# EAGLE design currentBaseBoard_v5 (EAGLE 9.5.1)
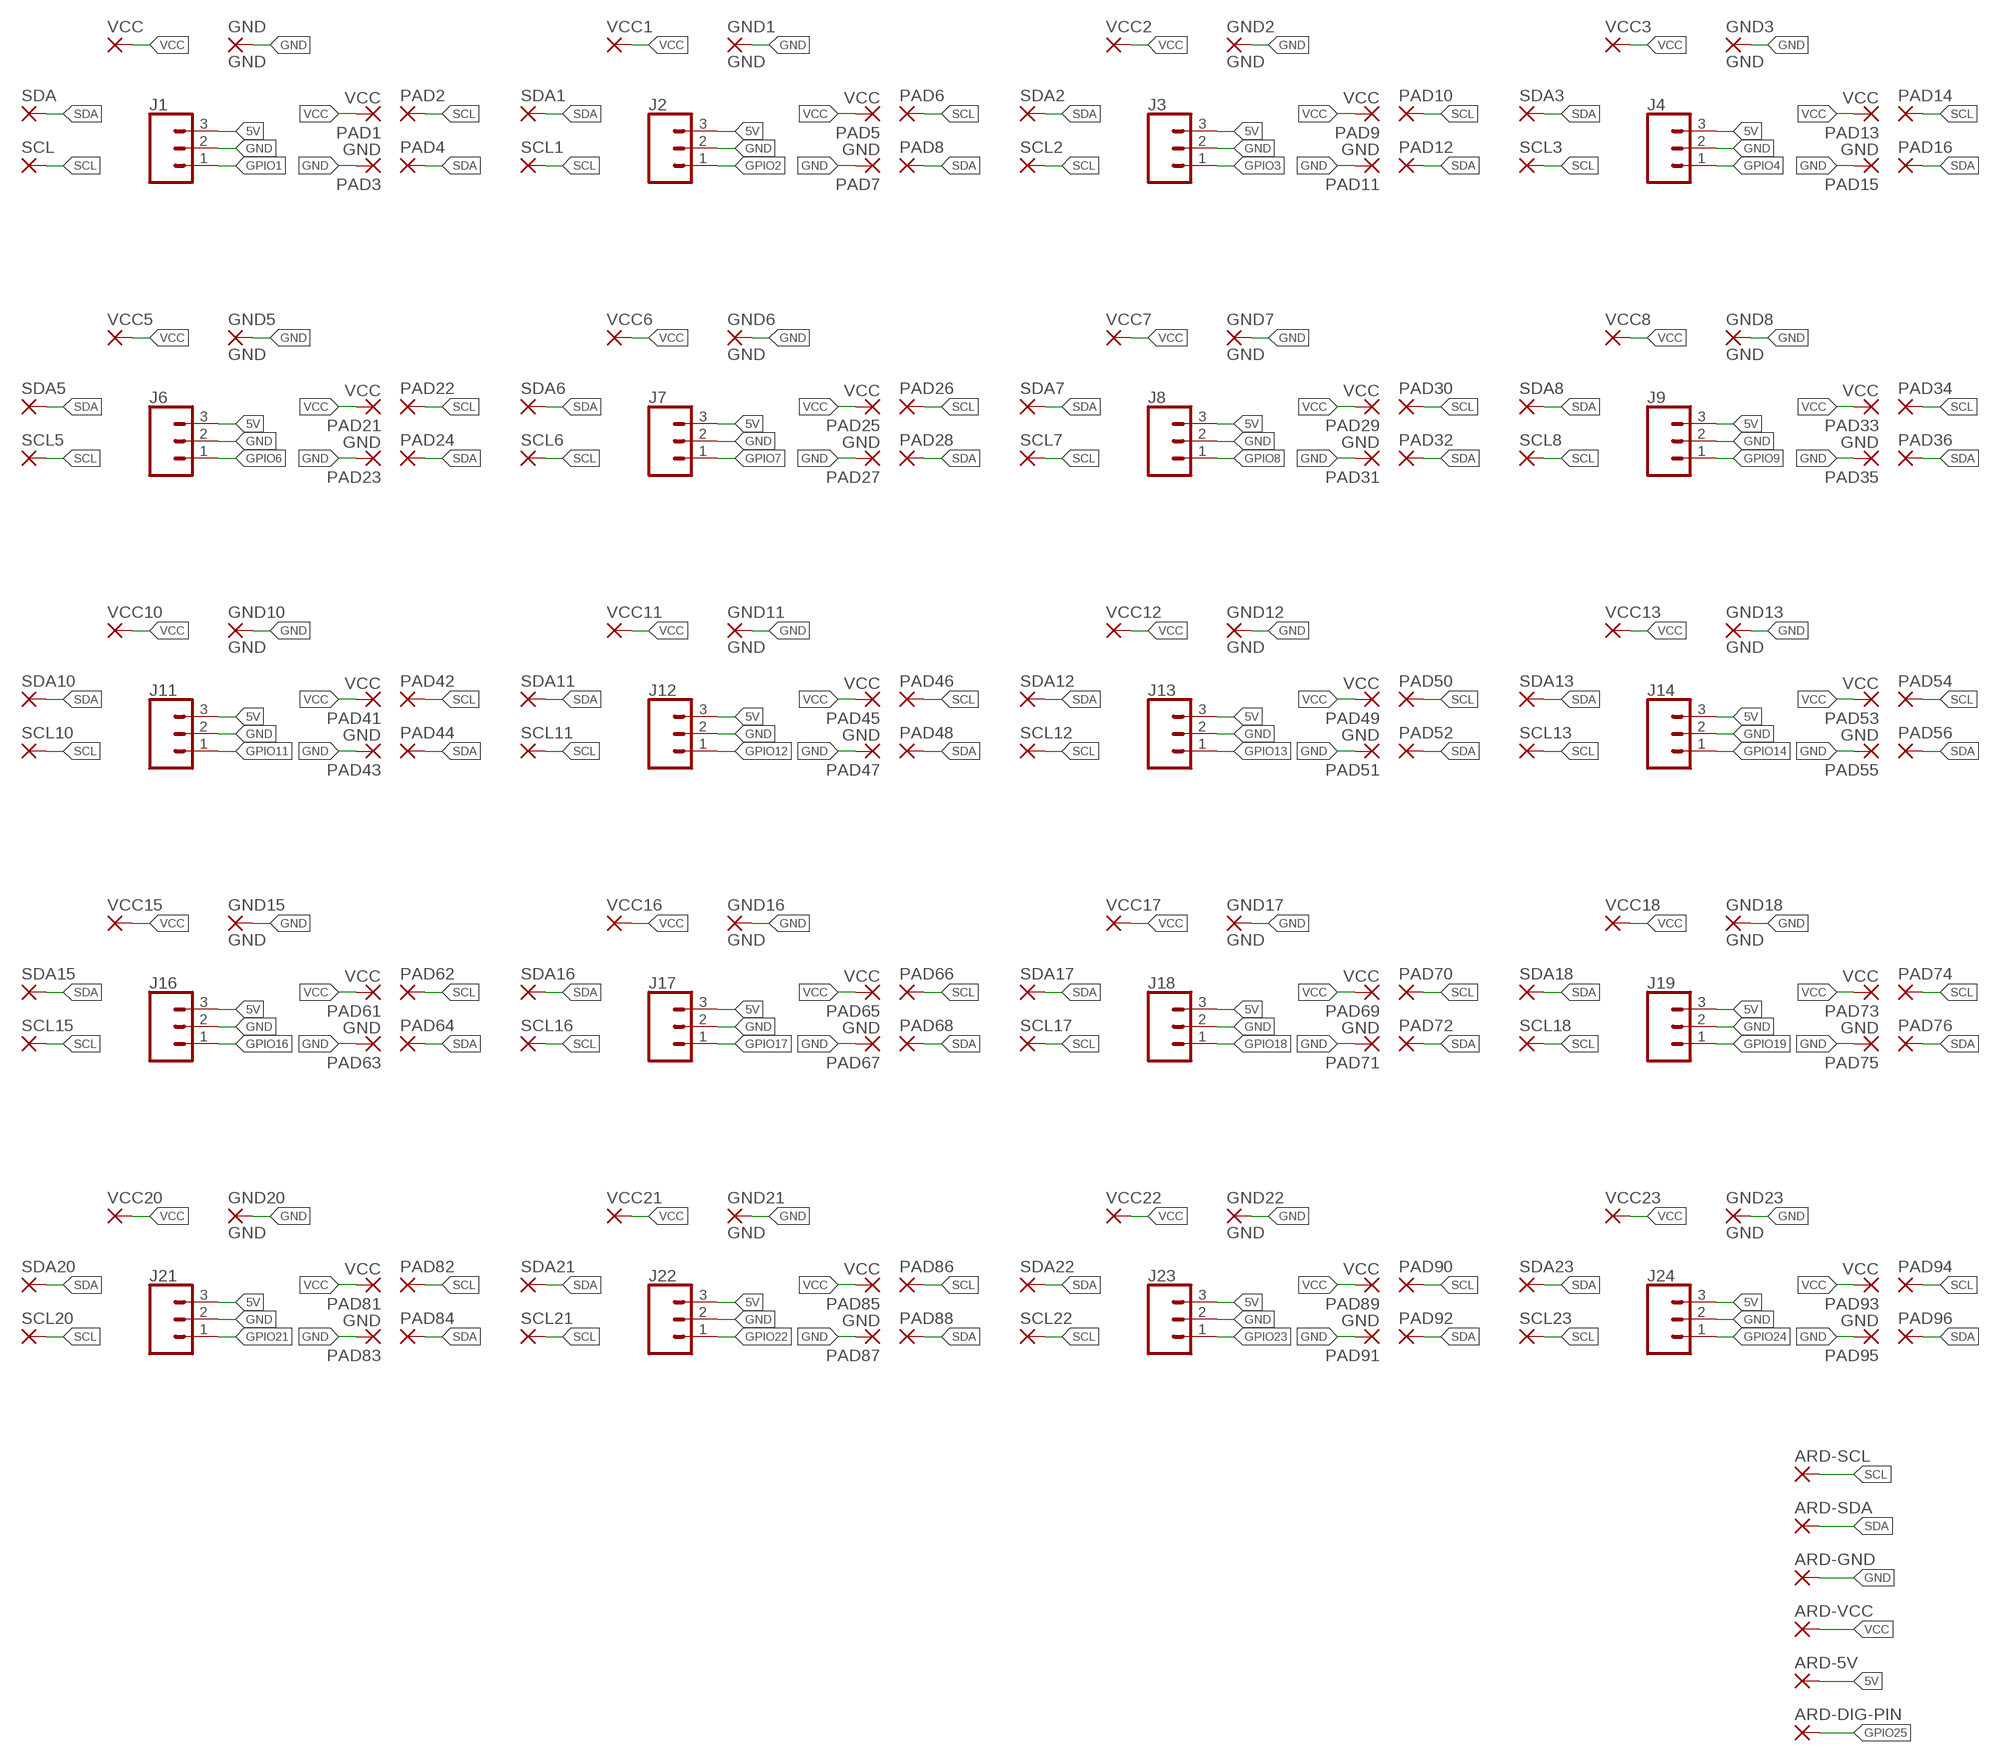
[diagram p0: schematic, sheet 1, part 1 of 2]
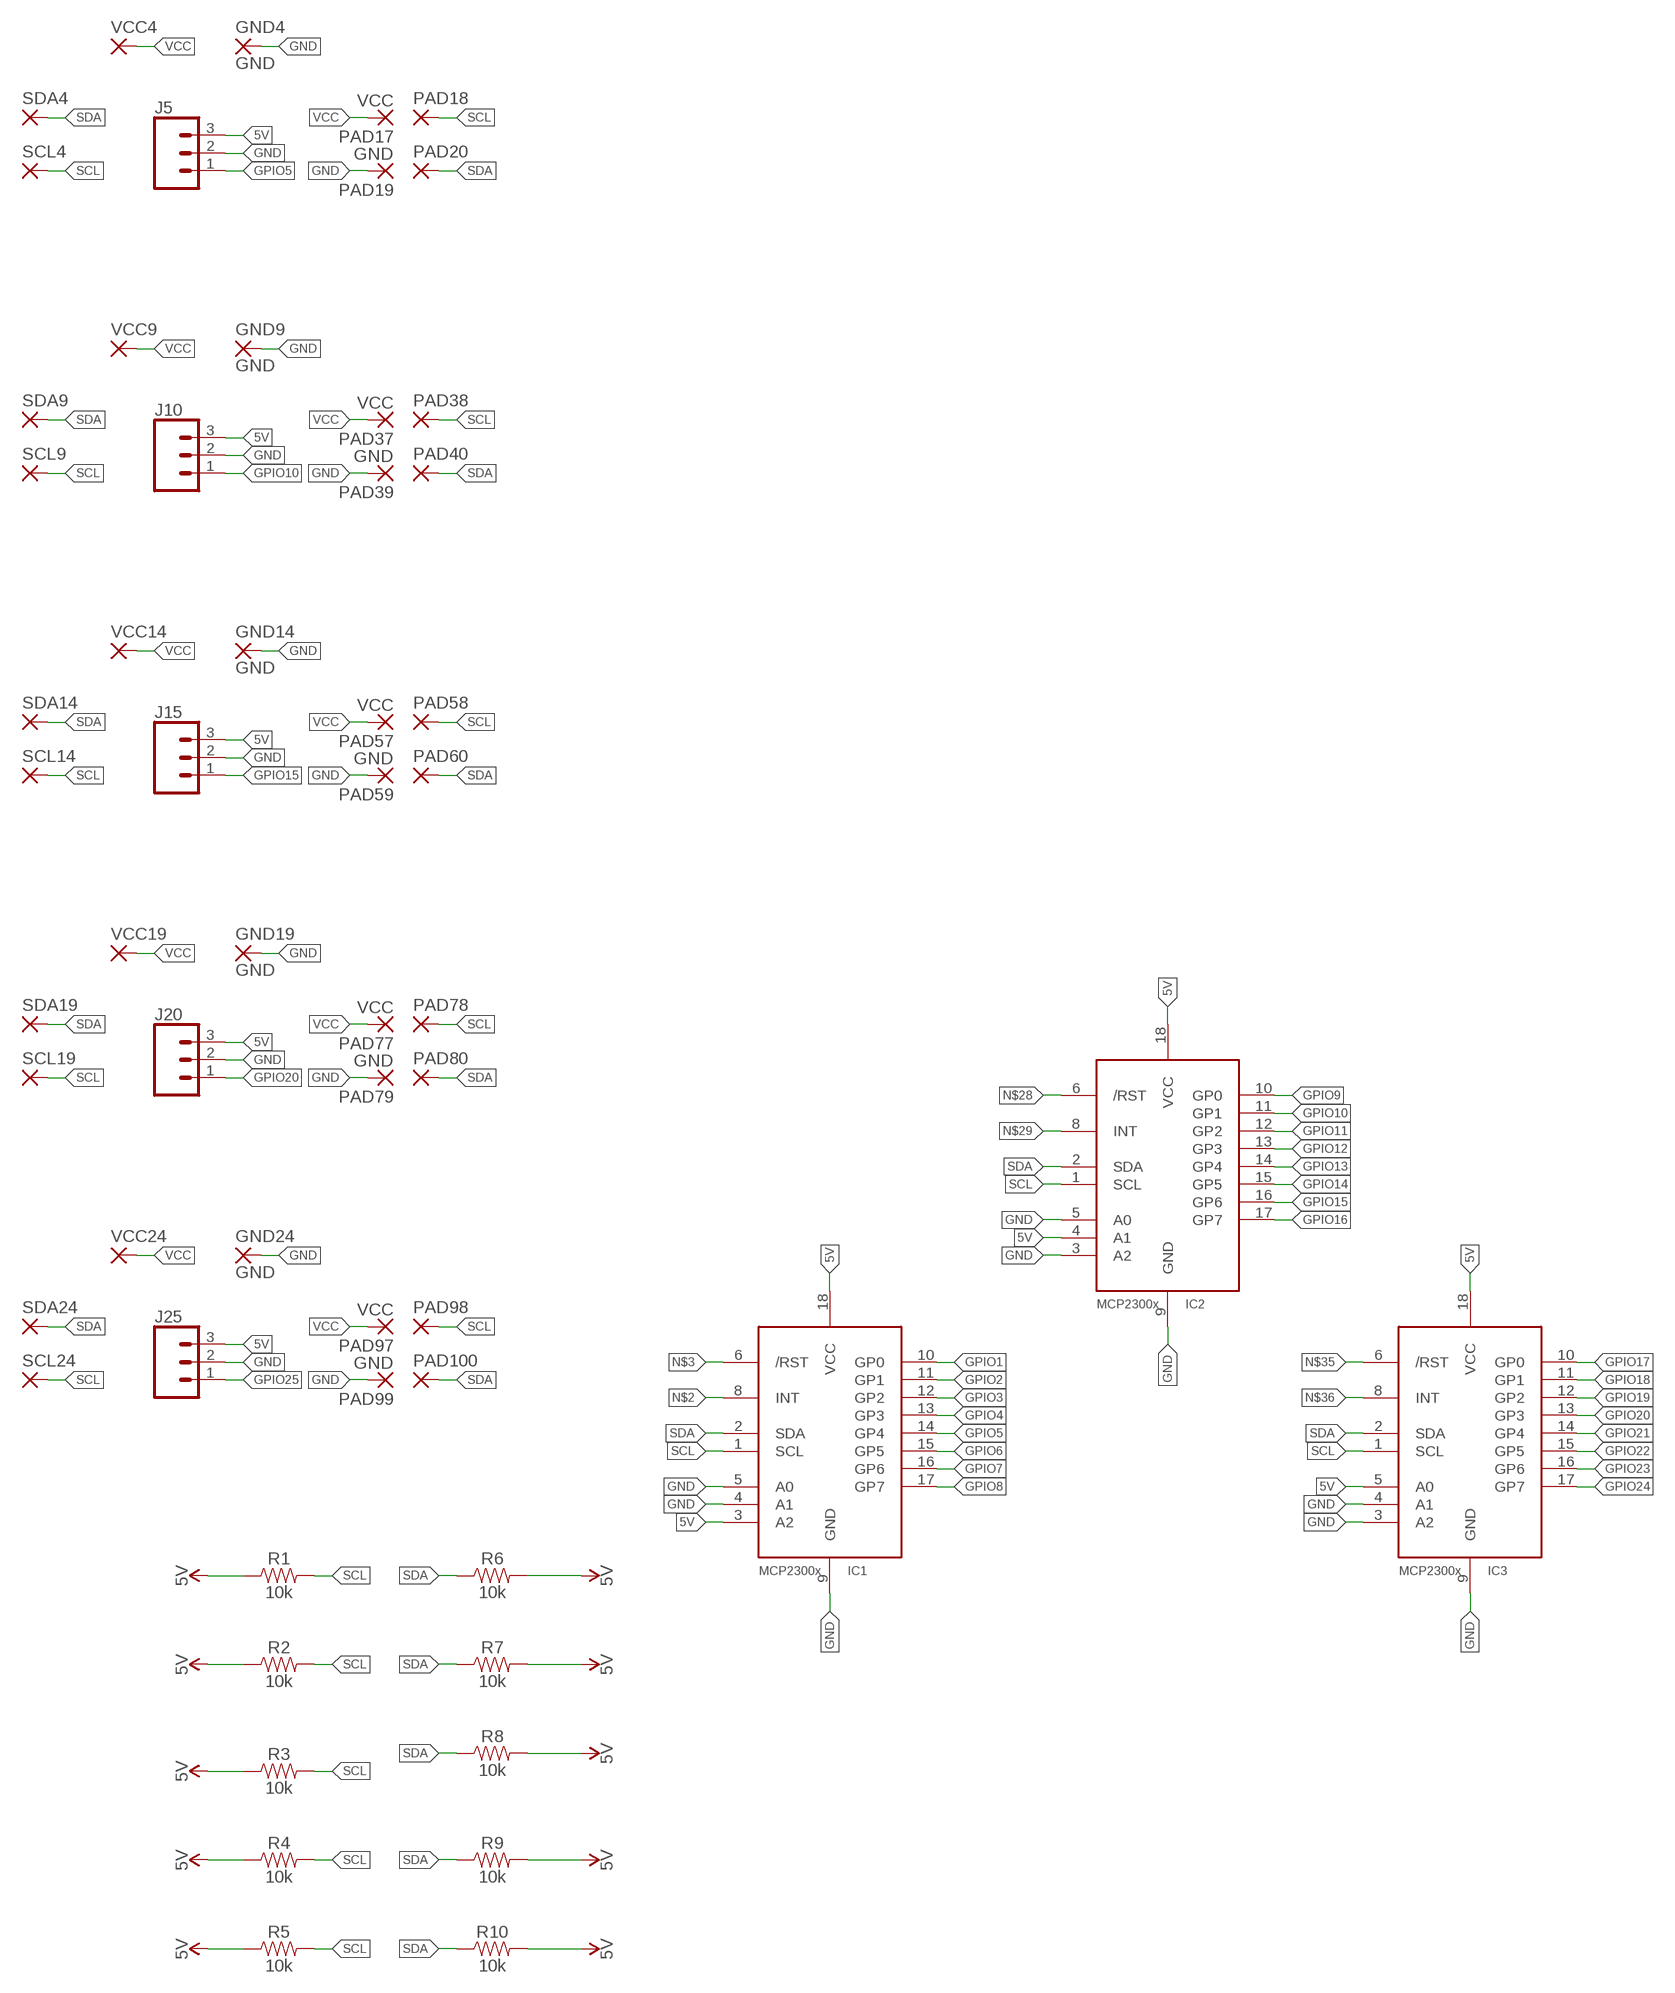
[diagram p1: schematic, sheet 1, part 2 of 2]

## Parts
ARD-5V  2,15/1,0  [2,15/1,0]
ARD-DIG-PIN  2,15/1,0  [2,15/1,0]
ARD-GND  2,15/1,0  [2,15/1,0]
ARD-SCL  2,15/1,0  [2,15/1,0]
ARD-SDA  2,15/1,0  [2,15/1,0]
ARD-VCC  2,15/1,0  [2,15/1,0]
GND  GND  2,15/1,0  [2,15/1,0]
GND1  GND  2,15/1,0  [2,15/1,0]
GND2  GND  2,15/1,0  [2,15/1,0]
GND3  GND  2,15/1,0  [2,15/1,0]
GND4  GND  2,15/1,0  [2,15/1,0]
GND5  GND  2,15/1,0  [2,15/1,0]
GND6  GND  2,15/1,0  [2,15/1,0]
GND7  GND  2,15/1,0  [2,15/1,0]
GND8  GND  2,15/1,0  [2,15/1,0]
GND9  GND  2,15/1,0  [2,15/1,0]
GND10  GND  2,15/1,0  [2,15/1,0]
GND11  GND  2,15/1,0  [2,15/1,0]
GND12  GND  2,15/1,0  [2,15/1,0]
GND13  GND  2,15/1,0  [2,15/1,0]
GND14  GND  2,15/1,0  [2,15/1,0]
GND15  GND  2,15/1,0  [2,15/1,0]
GND16  GND  2,15/1,0  [2,15/1,0]
GND17  GND  2,15/1,0  [2,15/1,0]
GND18  GND  2,15/1,0  [2,15/1,0]
GND19  GND  2,15/1,0  [2,15/1,0]
GND20  GND  2,15/1,0  [2,15/1,0]
GND21  GND  2,15/1,0  [2,15/1,0]
GND22  GND  2,15/1,0  [2,15/1,0]
GND23  GND  2,15/1,0  [2,15/1,0]
GND24  GND  2,15/1,0  [2,15/1,0]
IC1  MCP23008/P  [DIL18]
IC2  MCP23008/P  [DIL18]
IC3  MCP23008/P  [DIL18]
J1  CONN_03  [1X03]
J2  CONN_03  [1X03]
J3  CONN_03  [1X03]
J4  CONN_03  [1X03]
J5  CONN_03  [1X03]
J6  CONN_03  [1X03]
J7  CONN_03  [1X03]
J8  CONN_03  [1X03]
J9  CONN_03  [1X03]
J10  CONN_03  [1X03]
J11  CONN_03  [1X03]
J12  CONN_03  [1X03]
J13  CONN_03  [1X03]
J14  CONN_03  [1X03]
J15  CONN_03  [1X03]
J16  CONN_03  [1X03]
J17  CONN_03  [1X03]
J18  CONN_03  [1X03]
J19  CONN_03  [1X03]
J20  CONN_03  [1X03]
J21  CONN_03  [1X03]
J22  CONN_03  [1X03]
J23  CONN_03  [1X03]
J24  CONN_03  [1X03]
J25  CONN_03  [1X03]
PAD1  VCC  2,15/1,0  [2,15/1,0]
PAD2  2,15/1,0  [2,15/1,0]
PAD3  GND  2,15/1,0  [2,15/1,0]
PAD4  2,15/1,0  [2,15/1,0]
PAD5  VCC  2,15/1,0  [2,15/1,0]
PAD6  2,15/1,0  [2,15/1,0]
PAD7  GND  2,15/1,0  [2,15/1,0]
PAD8  2,15/1,0  [2,15/1,0]
PAD9  VCC  2,15/1,0  [2,15/1,0]
PAD10  2,15/1,0  [2,15/1,0]
PAD11  GND  2,15/1,0  [2,15/1,0]
PAD12  2,15/1,0  [2,15/1,0]
PAD13  VCC  2,15/1,0  [2,15/1,0]
PAD14  2,15/1,0  [2,15/1,0]
PAD15  GND  2,15/1,0  [2,15/1,0]
PAD16  2,15/1,0  [2,15/1,0]
PAD17  VCC  2,15/1,0  [2,15/1,0]
PAD18  2,15/1,0  [2,15/1,0]
PAD19  GND  2,15/1,0  [2,15/1,0]
PAD20  2,15/1,0  [2,15/1,0]
PAD21  VCC  2,15/1,0  [2,15/1,0]
PAD22  2,15/1,0  [2,15/1,0]
PAD23  GND  2,15/1,0  [2,15/1,0]
PAD24  2,15/1,0  [2,15/1,0]
PAD25  VCC  2,15/1,0  [2,15/1,0]
PAD26  2,15/1,0  [2,15/1,0]
PAD27  GND  2,15/1,0  [2,15/1,0]
PAD28  2,15/1,0  [2,15/1,0]
PAD29  VCC  2,15/1,0  [2,15/1,0]
PAD30  2,15/1,0  [2,15/1,0]
PAD31  GND  2,15/1,0  [2,15/1,0]
PAD32  2,15/1,0  [2,15/1,0]
PAD33  VCC  2,15/1,0  [2,15/1,0]
PAD34  2,15/1,0  [2,15/1,0]
PAD35  GND  2,15/1,0  [2,15/1,0]
PAD36  2,15/1,0  [2,15/1,0]
PAD37  VCC  2,15/1,0  [2,15/1,0]
PAD38  2,15/1,0  [2,15/1,0]
PAD39  GND  2,15/1,0  [2,15/1,0]
PAD40  2,15/1,0  [2,15/1,0]
PAD41  VCC  2,15/1,0  [2,15/1,0]
PAD42  2,15/1,0  [2,15/1,0]
PAD43  GND  2,15/1,0  [2,15/1,0]
PAD44  2,15/1,0  [2,15/1,0]
PAD45  VCC  2,15/1,0  [2,15/1,0]
PAD46  2,15/1,0  [2,15/1,0]
PAD47  GND  2,15/1,0  [2,15/1,0]
PAD48  2,15/1,0  [2,15/1,0]
PAD49  VCC  2,15/1,0  [2,15/1,0]
PAD50  2,15/1,0  [2,15/1,0]
PAD51  GND  2,15/1,0  [2,15/1,0]
PAD52  2,15/1,0  [2,15/1,0]
PAD53  VCC  2,15/1,0  [2,15/1,0]
PAD54  2,15/1,0  [2,15/1,0]
PAD55  GND  2,15/1,0  [2,15/1,0]
PAD56  2,15/1,0  [2,15/1,0]
PAD57  VCC  2,15/1,0  [2,15/1,0]
PAD58  2,15/1,0  [2,15/1,0]
PAD59  GND  2,15/1,0  [2,15/1,0]
PAD60  2,15/1,0  [2,15/1,0]
PAD61  VCC  2,15/1,0  [2,15/1,0]
PAD62  2,15/1,0  [2,15/1,0]
PAD63  GND  2,15/1,0  [2,15/1,0]
PAD64  2,15/1,0  [2,15/1,0]
PAD65  VCC  2,15/1,0  [2,15/1,0]
PAD66  2,15/1,0  [2,15/1,0]
PAD67  GND  2,15/1,0  [2,15/1,0]
PAD68  2,15/1,0  [2,15/1,0]
PAD69  VCC  2,15/1,0  [2,15/1,0]
PAD70  2,15/1,0  [2,15/1,0]
PAD71  GND  2,15/1,0  [2,15/1,0]
PAD72  2,15/1,0  [2,15/1,0]
PAD73  VCC  2,15/1,0  [2,15/1,0]
PAD74  2,15/1,0  [2,15/1,0]
PAD75  GND  2,15/1,0  [2,15/1,0]
PAD76  2,15/1,0  [2,15/1,0]
PAD77  VCC  2,15/1,0  [2,15/1,0]
PAD78  2,15/1,0  [2,15/1,0]
PAD79  GND  2,15/1,0  [2,15/1,0]
PAD80  2,15/1,0  [2,15/1,0]
PAD81  VCC  2,15/1,0  [2,15/1,0]
PAD82  2,15/1,0  [2,15/1,0]
PAD83  GND  2,15/1,0  [2,15/1,0]
PAD84  2,15/1,0  [2,15/1,0]
PAD85  VCC  2,15/1,0  [2,15/1,0]
PAD86  2,15/1,0  [2,15/1,0]
PAD87  GND  2,15/1,0  [2,15/1,0]
PAD88  2,15/1,0  [2,15/1,0]
PAD89  VCC  2,15/1,0  [2,15/1,0]
PAD90  2,15/1,0  [2,15/1,0]
PAD91  GND  2,15/1,0  [2,15/1,0]
PAD92  2,15/1,0  [2,15/1,0]
PAD93  VCC  2,15/1,0  [2,15/1,0]
PAD94  2,15/1,0  [2,15/1,0]
PAD95  GND  2,15/1,0  [2,15/1,0]
PAD96  2,15/1,0  [2,15/1,0]
PAD97  VCC  2,15/1,0  [2,15/1,0]
PAD98  2,15/1,0  [2,15/1,0]
PAD99  GND  2,15/1,0  [2,15/1,0]
PAD100  2,15/1,0  [2,15/1,0]
R1  10k  10KOHM-HORIZ-1/4W-1%  [AXIAL-0.3]
R2  10k  10KOHM-HORIZ-1/4W-1%  [AXIAL-0.3]
R3  10k  10KOHM-HORIZ-1/4W-1%  [AXIAL-0.3]
R4  10k  10KOHM-HORIZ-1/4W-1%  [AXIAL-0.3]
R5  10k  10KOHM-HORIZ-1/4W-1%  [AXIAL-0.3]
R6  10k  10KOHM-HORIZ-1/4W-1%  [AXIAL-0.3]
R7  10k  10KOHM-HORIZ-1/4W-1%  [AXIAL-0.3]
R8  10k  10KOHM-HORIZ-1/4W-1%  [AXIAL-0.3]
R9  10k  10KOHM-HORIZ-1/4W-1%  [AXIAL-0.3]
R10  10k  10KOHM-HORIZ-1/4W-1%  [AXIAL-0.3]
SCL  2,15/1,0  [2,15/1,0]
SCL1  2,15/1,0  [2,15/1,0]
SCL2  2,15/1,0  [2,15/1,0]
SCL3  2,15/1,0  [2,15/1,0]
SCL4  2,15/1,0  [2,15/1,0]
SCL5  2,15/1,0  [2,15/1,0]
SCL6  2,15/1,0  [2,15/1,0]
SCL7  2,15/1,0  [2,15/1,0]
SCL8  2,15/1,0  [2,15/1,0]
SCL9  2,15/1,0  [2,15/1,0]
SCL10  2,15/1,0  [2,15/1,0]
SCL11  2,15/1,0  [2,15/1,0]
SCL12  2,15/1,0  [2,15/1,0]
SCL13  2,15/1,0  [2,15/1,0]
SCL14  2,15/1,0  [2,15/1,0]
SCL15  2,15/1,0  [2,15/1,0]
SCL16  2,15/1,0  [2,15/1,0]
SCL17  2,15/1,0  [2,15/1,0]
SCL18  2,15/1,0  [2,15/1,0]
SCL19  2,15/1,0  [2,15/1,0]
SCL20  2,15/1,0  [2,15/1,0]
SCL21  2,15/1,0  [2,15/1,0]
SCL22  2,15/1,0  [2,15/1,0]
SCL23  2,15/1,0  [2,15/1,0]
SCL24  2,15/1,0  [2,15/1,0]
SDA  2,15/1,0  [2,15/1,0]
SDA1  2,15/1,0  [2,15/1,0]
SDA2  2,15/1,0  [2,15/1,0]
SDA3  2,15/1,0  [2,15/1,0]
SDA4  2,15/1,0  [2,15/1,0]
SDA5  2,15/1,0  [2,15/1,0]
SDA6  2,15/1,0  [2,15/1,0]
SDA7  2,15/1,0  [2,15/1,0]
SDA8  2,15/1,0  [2,15/1,0]
SDA9  2,15/1,0  [2,15/1,0]
SDA10  2,15/1,0  [2,15/1,0]
SDA11  2,15/1,0  [2,15/1,0]
SDA12  2,15/1,0  [2,15/1,0]
SDA13  2,15/1,0  [2,15/1,0]
SDA14  2,15/1,0  [2,15/1,0]
SDA15  2,15/1,0  [2,15/1,0]
SDA16  2,15/1,0  [2,15/1,0]
SDA17  2,15/1,0  [2,15/1,0]
SDA18  2,15/1,0  [2,15/1,0]
SDA19  2,15/1,0  [2,15/1,0]
SDA20  2,15/1,0  [2,15/1,0]
SDA21  2,15/1,0  [2,15/1,0]
SDA22  2,15/1,0  [2,15/1,0]
SDA23  2,15/1,0  [2,15/1,0]
SDA24  2,15/1,0  [2,15/1,0]
VCC  2,15/1,0  [2,15/1,0]
VCC1  2,15/1,0  [2,15/1,0]
VCC2  2,15/1,0  [2,15/1,0]
VCC3  2,15/1,0  [2,15/1,0]
VCC4  2,15/1,0  [2,15/1,0]
VCC5  2,15/1,0  [2,15/1,0]
VCC6  2,15/1,0  [2,15/1,0]
VCC7  2,15/1,0  [2,15/1,0]
VCC8  2,15/1,0  [2,15/1,0]
VCC9  2,15/1,0  [2,15/1,0]
VCC10  2,15/1,0  [2,15/1,0]
VCC11  2,15/1,0  [2,15/1,0]
VCC12  2,15/1,0  [2,15/1,0]
VCC13  2,15/1,0  [2,15/1,0]
VCC14  2,15/1,0  [2,15/1,0]
VCC15  2,15/1,0  [2,15/1,0]
VCC16  2,15/1,0  [2,15/1,0]
VCC17  2,15/1,0  [2,15/1,0]
VCC18  2,15/1,0  [2,15/1,0]
VCC19  2,15/1,0  [2,15/1,0]
VCC20  2,15/1,0  [2,15/1,0]
VCC21  2,15/1,0  [2,15/1,0]
VCC22  2,15/1,0  [2,15/1,0]
VCC23  2,15/1,0  [2,15/1,0]
VCC24  2,15/1,0  [2,15/1,0]

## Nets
5V: ARD-5V.1(P) IC1.3(A2) IC1.18(VCC) IC2.4(A1) IC2.18(VCC) IC3.5(A0) IC3.18(VCC) J1.3 J2.3 J3.3 J4.3 J5.3 J6.3 J7.3 J8.3 J9.3 J10.3 J11.3 J12.3 J13.3 J14.3 J15.3 J16.3 J17.3 J18.3 J19.3 J20.3 J21.3 J22.3 J23.3 J24.3 J25.3 R1.P$1 R2.P$1 R3.P$1 R4.P$1 R5.P$1 R6.P$2 R7.P$2 R8.P$2 R9.P$2 R10.P$2
GND: ARD-GND.1(P) GND1.1(P) GND2.1(P) GND3.1(P) GND4.1(P) GND5.1(P) GND6.1(P) GND7.1(P) GND8.1(P) GND9.1(P) GND10.1(P) GND11.1(P) GND12.1(P) GND13.1(P) GND14.1(P) GND15.1(P) GND16.1(P) GND17.1(P) GND18.1(P) GND19.1(P) GND20.1(P) GND21.1(P) GND22.1(P) GND23.1(P) GND24.1(P) GND.1(P) IC1.4(A1) IC1.5(A0) IC1.9(GND) IC2.3(A2) IC2.5(A0) IC2.9(GND) IC3.3(A2) IC3.4(A1) IC3.9(GND) J1.2 J2.2 J3.2 J4.2 J5.2 J6.2 J7.2 J8.2 J9.2 J10.2 J11.2 J12.2 J13.2 J14.2 J15.2 J16.2 J17.2 J18.2 J19.2 J20.2 J21.2 J22.2 J23.2 J24.2 J25.2 PAD3.1(P) PAD7.1(P) PAD11.1(P) PAD15.1(P) PAD19.1(P) PAD23.1(P) PAD27.1(P) PAD31.1(P) PAD35.1(P) PAD39.1(P) PAD43.1(P) PAD47.1(P) PAD51.1(P) PAD55.1(P) PAD59.1(P) PAD63.1(P) PAD67.1(P) PAD71.1(P) PAD75.1(P) PAD79.1(P) PAD83.1(P) PAD87.1(P) PAD91.1(P) PAD95.1(P) PAD99.1(P)
GPIO1: IC1.10(GP0) J1.1
GPIO2: IC1.11(GP1) J2.1
GPIO3: IC1.12(GP2) J3.1
GPIO4: IC1.13(GP3) J4.1
GPIO5: IC1.14(GP4) J5.1
GPIO6: IC1.15(GP5) J6.1
GPIO7: IC1.16(GP6) J7.1
GPIO8: IC1.17(GP7) J8.1
GPIO9: IC2.10(GP0) J9.1
GPIO10: IC2.11(GP1) J10.1
GPIO11: IC2.12(GP2) J11.1
GPIO12: IC2.13(GP3) J12.1
GPIO13: IC2.14(GP4) J13.1
GPIO14: IC2.15(GP5) J14.1
GPIO15: IC2.16(GP6) J15.1
GPIO16: IC2.17(GP7) J16.1
GPIO17: IC3.10(GP0) J17.1
GPIO18: IC3.11(GP1) J18.1
GPIO19: IC3.12(GP2) J19.1
GPIO20: IC3.13(GP3) J20.1
GPIO21: IC3.14(GP4) J21.1
GPIO22: IC3.15(GP5) J22.1
GPIO23: IC3.16(GP6) J23.1
GPIO24: IC3.17(GP7) J24.1
GPIO25: ARD-DIG-PIN.1(P) J25.1
N$2: IC1.8(INT)
N$3: IC1.6(/RST)
N$28: IC2.6(/RST)
N$29: IC2.8(INT)
N$35: IC3.6(/RST)
N$36: IC3.8(INT)
SCL: ARD-SCL.1(P) IC1.1(SCL) IC2.1(SCL) IC3.1(SCL) PAD2.1(P) PAD6.1(P) PAD10.1(P) PAD14.1(P) PAD18.1(P) PAD22.1(P) PAD26.1(P) PAD30.1(P) PAD34.1(P) PAD38.1(P) PAD42.1(P) PAD46.1(P) PAD50.1(P) PAD54.1(P) PAD58.1(P) PAD62.1(P) PAD66.1(P) PAD70.1(P) PAD74.1(P) PAD78.1(P) PAD82.1(P) PAD86.1(P) PAD90.1(P) PAD94.1(P) PAD98.1(P) R1.P$2 R2.P$2 R3.P$2 R4.P$2 R5.P$2 SCL1.1(P) SCL2.1(P) SCL3.1(P) SCL4.1(P) SCL5.1(P) SCL6.1(P) SCL7.1(P) SCL8.1(P) SCL9.1(P) SCL10.1(P) SCL11.1(P) SCL12.1(P) SCL13.1(P) SCL14.1(P) SCL15.1(P) SCL16.1(P) SCL17.1(P) SCL18.1(P) SCL19.1(P) SCL20.1(P) SCL21.1(P) SCL22.1(P) SCL23.1(P) SCL24.1(P) SCL.1(P)
SDA: ARD-SDA.1(P) IC1.2(SDA) IC2.2(SDA) IC3.2(SDA) PAD4.1(P) PAD8.1(P) PAD12.1(P) PAD16.1(P) PAD20.1(P) PAD24.1(P) PAD28.1(P) PAD32.1(P) PAD36.1(P) PAD40.1(P) PAD44.1(P) PAD48.1(P) PAD52.1(P) PAD56.1(P) PAD60.1(P) PAD64.1(P) PAD68.1(P) PAD72.1(P) PAD76.1(P) PAD80.1(P) PAD84.1(P) PAD88.1(P) PAD92.1(P) PAD96.1(P) PAD100.1(P) R6.P$1 R7.P$1 R8.P$1 R9.P$1 R10.P$1 SDA1.1(P) SDA2.1(P) SDA3.1(P) SDA4.1(P) SDA5.1(P) SDA6.1(P) SDA7.1(P) SDA8.1(P) SDA9.1(P) SDA10.1(P) SDA11.1(P) SDA12.1(P) SDA13.1(P) SDA14.1(P) SDA15.1(P) SDA16.1(P) SDA17.1(P) SDA18.1(P) SDA19.1(P) SDA20.1(P) SDA21.1(P) SDA22.1(P) SDA23.1(P) SDA24.1(P) SDA.1(P)
VCC: ARD-VCC.1(P) PAD1.1(P) PAD5.1(P) PAD9.1(P) PAD13.1(P) PAD17.1(P) PAD21.1(P) PAD25.1(P) PAD29.1(P) PAD33.1(P) PAD37.1(P) PAD41.1(P) PAD45.1(P) PAD49.1(P) PAD53.1(P) PAD57.1(P) PAD61.1(P) PAD65.1(P) PAD69.1(P) PAD73.1(P) PAD77.1(P) PAD81.1(P) PAD85.1(P) PAD89.1(P) PAD93.1(P) PAD97.1(P) VCC1.1(P) VCC2.1(P) VCC3.1(P) VCC4.1(P) VCC5.1(P) VCC6.1(P) VCC7.1(P) VCC8.1(P) VCC9.1(P) VCC10.1(P) VCC11.1(P) VCC12.1(P) VCC13.1(P) VCC14.1(P) VCC15.1(P) VCC16.1(P) VCC17.1(P) VCC18.1(P) VCC19.1(P) VCC20.1(P) VCC21.1(P) VCC22.1(P) VCC23.1(P) VCC24.1(P) VCC.1(P)

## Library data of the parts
ARD-5V ARD-DIG-PIN ARD-GND ARD-SCL ARD-SDA ARD-VCC GND GND1-GND24 PAD1-PAD100 SCL SCL1-SCL24 SDA SDA1-SDA24 VCC VCC1-VCC24 = wirepad:2,15/1,0: THROUGH-HOLE PAD
IC1-IC3 = adafruit:MCP23008: MCP23008 Inexpensive i2c i/o expander - 8 general purpose i/o pins with optional pullups
J1-J25 = SparkFun-Connectors:CONN_03: Multi connection point. Often used as Generic Header-pin footprint for 0.1 inch spaced/style header connections On any of the 0.1 inch spaced packages, you can populate with these: Break Away Headers - Straight (PRT-00116) Break Away Male Headers - Right Angle (PRT-00553) Female Headers (PRT-00115)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
R1-R10 = SparkFun-Resistors:10KOHM: 10kΩ resistor; PROD_ID: RES-12183

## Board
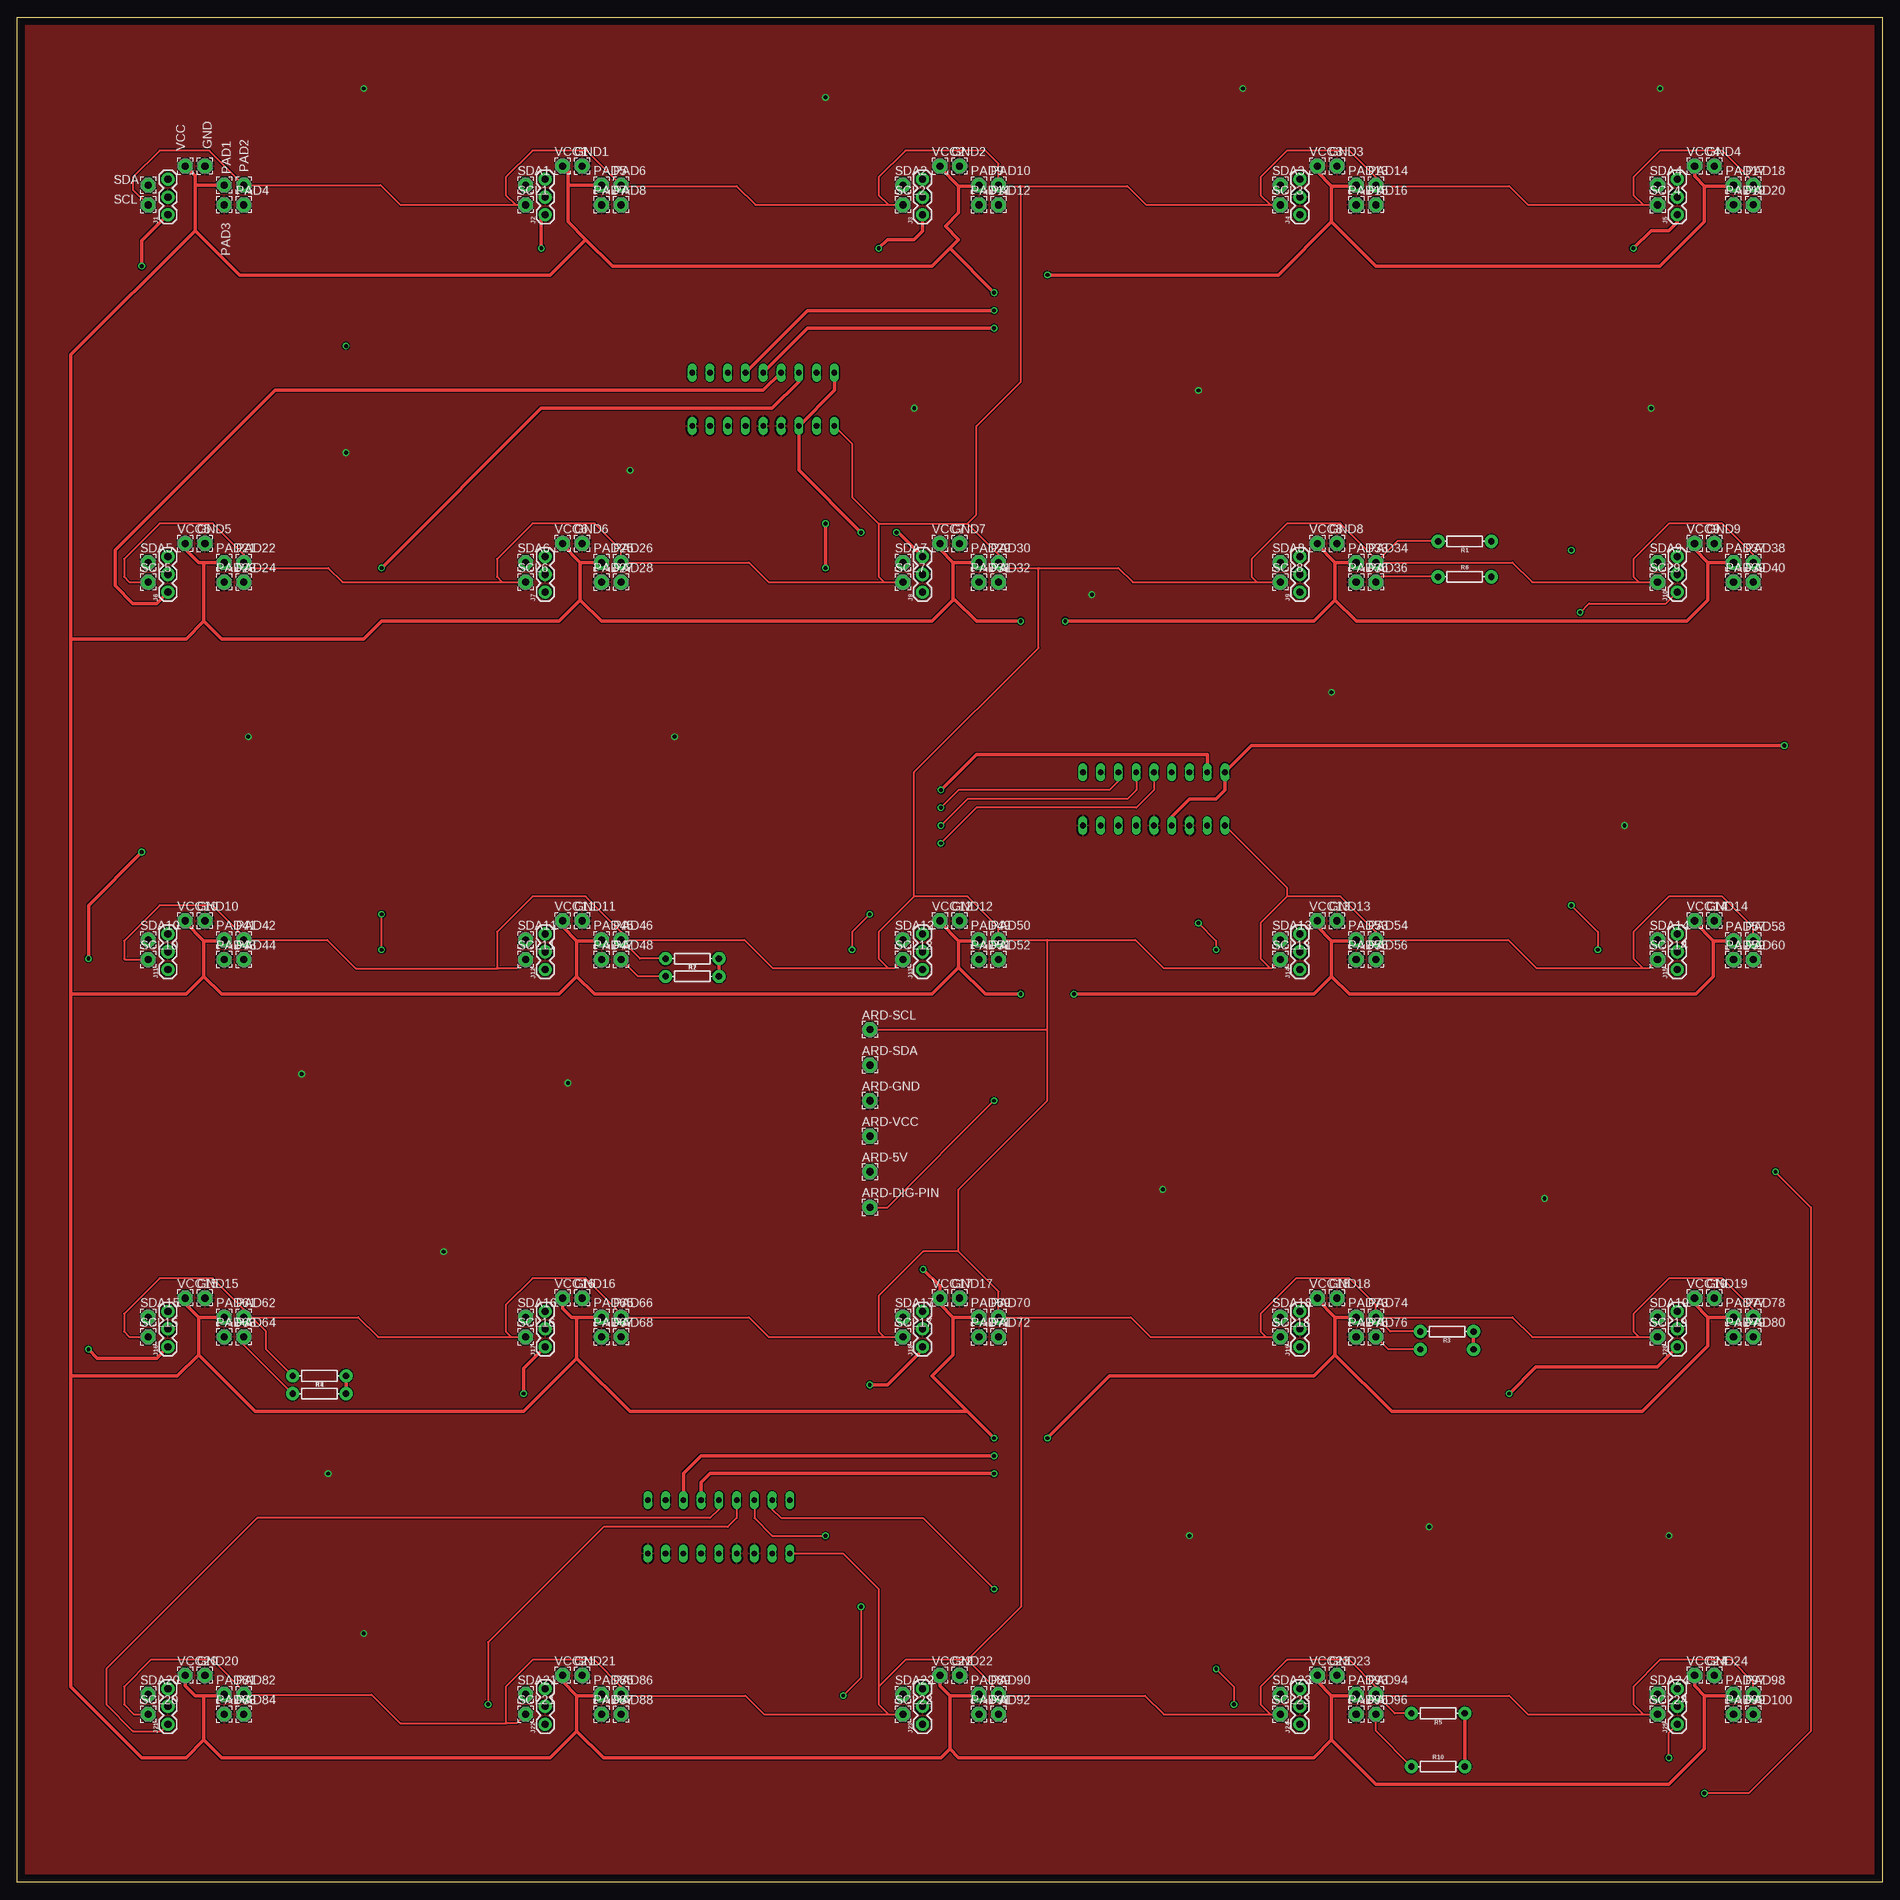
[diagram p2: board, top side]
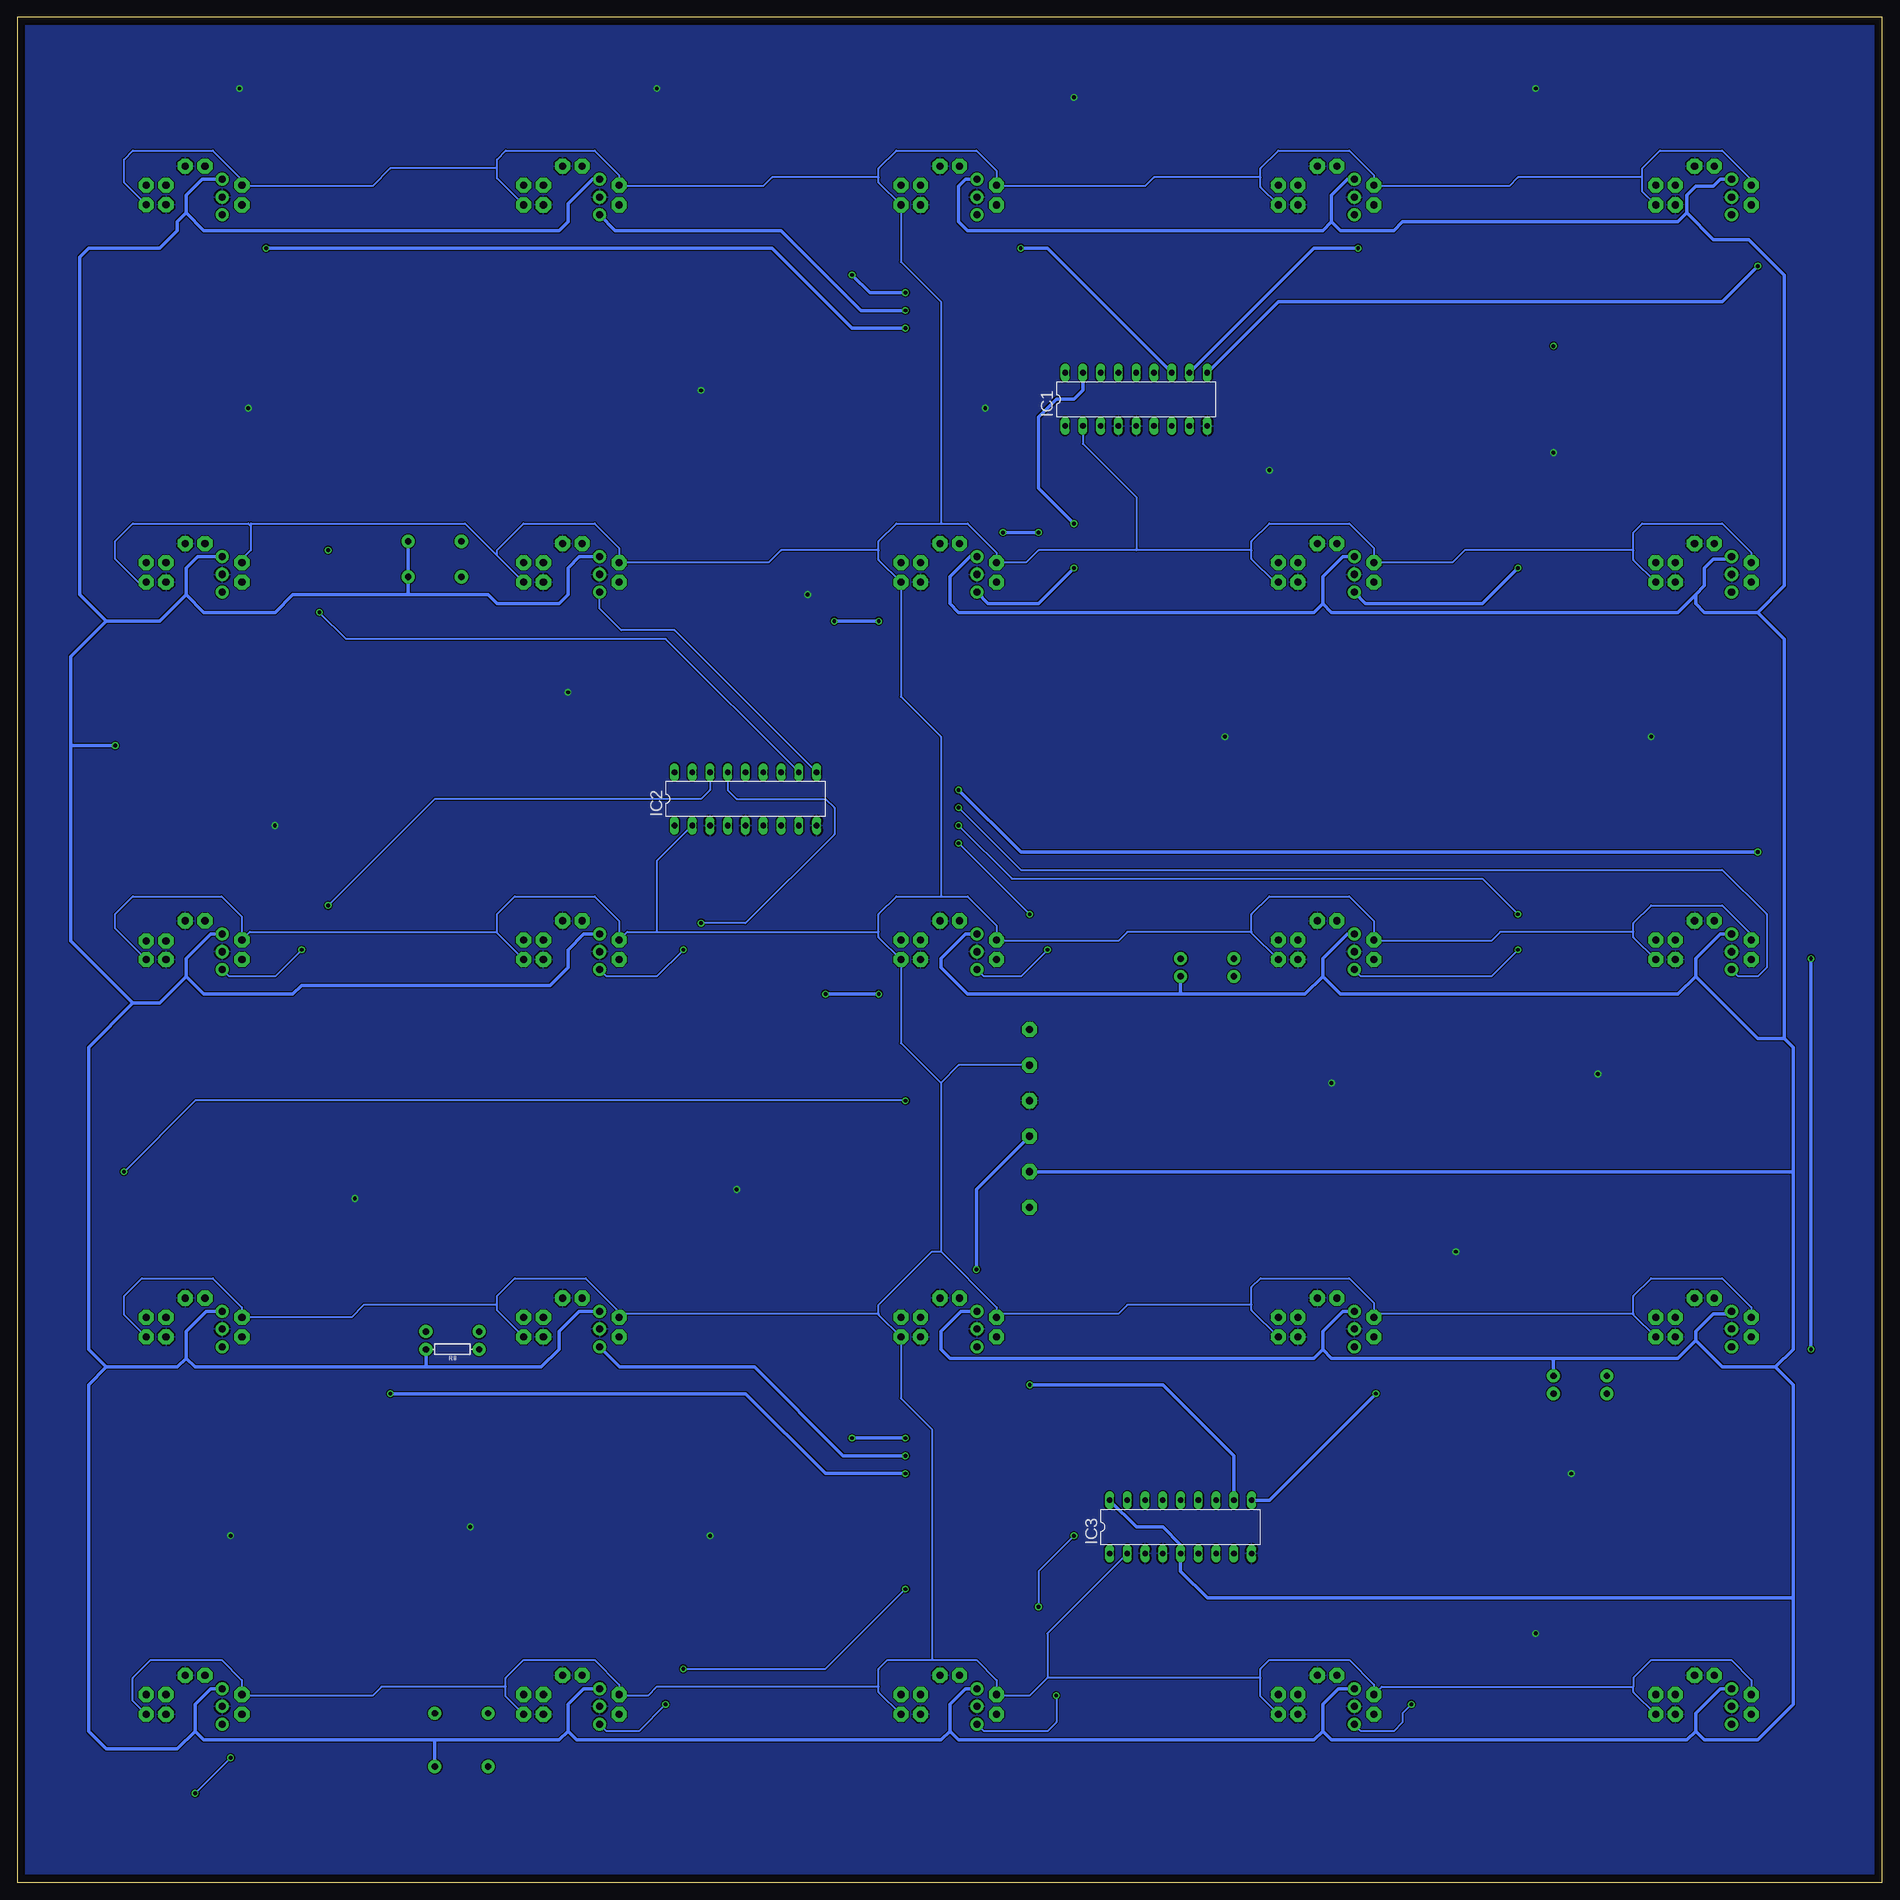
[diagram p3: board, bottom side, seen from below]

Size 266.7 x 266.7 mm. Coordinates in mm from the lower left corner, seen from the top.
Outline: 0,0 0,266.7 266.7,266.7 266.7,0 0,0
Copper layers (1*16): Top 0.035mm / dielectric 1.5mm / Bottom 0.035mm
Design rules "default": minimum track width 6mil, minimum drill 0.35mm, track to track 6mil, track to pad 6mil, pad to pad 6mil, via to via 6mil, smd to smd 6mil, copper to edge 40mil, drill to drill 6mil, minimum pad ring 10mil, minimum via ring 8mil, stop-mask expansion 4mil, vias tented up to drill 0mil, thermal gap 10mil

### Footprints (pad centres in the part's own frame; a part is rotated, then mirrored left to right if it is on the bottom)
2,15/1,0 = drill 1.016 pad 2.159 octagon: 1 0,0
DIL18 = drill 0.813 long: 1 -10.16,-3.81; 2 -7.62,-3.81; 3 -5.08,-3.81; 4 -2.54,-3.81; 5 0,-3.81; 6 2.54,-3.81; 7 5.08,-3.81; 8 7.62,-3.81; 9 10.16,-3.81; 10 10.16,3.81; 11 7.62,3.81; 12 5.08,3.81; 13 2.54,3.81; 14 0,3.81; 15 -2.54,3.81; 16 -5.08,3.81; 17 -7.62,3.81; 18 -10.16,3.81
1X03 = drill 1.016 pad 1.88: 1 0,0; 2 2.54,0; 3 5.08,0
AXIAL-0.3 = drill 0.9 pad 1.88: P$1 -3.81,0; P$2 3.81,0

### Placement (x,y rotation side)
ARD-5V  121.92,101.6 0 top
ARD-DIG-PIN  121.92,96.52 0 top
ARD-GND  121.92,111.76 0 top
ARD-SCL  121.92,121.92 0 top
ARD-SDA  121.92,116.84 0 top
ARD-VCC  121.92,106.68 0 top
GND  26.81,245.45 0 top
GND1  80.79,245.45 0 top
GND2  134.76,245.45 0 top
GND3  188.74,245.45 0 top
GND4  242.71,245.45 0 top
GND5  26.81,191.47 0 top
GND6  80.79,191.47 0 top
GND7  134.76,191.47 0 top
GND8  188.74,191.47 0 top
GND9  242.71,191.47 0 top
GND10  26.81,137.5 0 top
GND11  80.79,137.5 0 top
GND12  134.76,137.5 0 top
GND13  188.74,137.5 0 top
GND14  242.71,137.5 0 top
GND15  26.81,83.52 0 top
GND16  80.79,83.52 0 top
GND17  134.76,83.52 0 top
GND18  188.74,83.52 0 top
GND19  242.71,83.52 0 top
GND20  26.81,29.55 0 top
GND21  80.79,29.55 0 top
GND22  134.76,29.55 0 top
GND23  188.74,29.55 0 top
GND24  242.71,29.55 0 top
IC1  106.68,212.09 0 bottom
IC2  162.56,154.94 0 bottom
IC3  100.33,50.8 0 bottom
J1  21.52,238.48 90 top
J2  75.49,238.48 90 top
J3  129.47,238.48 90 top
J4  183.44,238.48 90 top
J5  237.42,238.48 90 top
J6  21.52,184.5 90 top
J7  75.49,184.5 90 top
J8  129.47,184.5 90 top
J9  183.44,184.5 90 top
J10  237.42,184.5 90 top
J11  21.52,130.53 90 top
J12  75.49,130.53 90 top
J13  129.47,130.53 90 top
J14  183.44,130.53 90 top
J15  237.42,130.53 90 top
J16  21.52,76.55 90 top
J17  75.49,76.55 90 top
J18  129.47,76.55 90 top
J19  183.44,76.55 90 top
J20  237.42,76.55 90 top
J21  21.52,22.58 90 top
J22  75.49,22.58 90 top
J23  129.47,22.58 90 top
J24  183.44,22.58 90 top
J25  237.42,22.58 90 top
PAD1  29.56,242.71 0 top
PAD2  32.38,242.71 0 top
PAD3  29.56,239.89 0 top
PAD4  32.38,239.89 0 top
PAD5  83.53,242.71 0 top
PAD6  86.35,242.71 0 top
PAD7  83.53,239.89 0 top
PAD8  86.35,239.89 0 top
PAD9  137.51,242.71 0 top
PAD10  140.33,242.71 0 top
PAD11  137.51,239.89 0 top
PAD12  140.33,239.89 0 top
PAD13  191.48,242.71 0 top
PAD14  194.3,242.71 0 top
PAD15  191.48,239.89 0 top
PAD16  194.3,239.89 0 top
PAD17  245.46,242.71 0 top
PAD18  248.28,242.71 0 top
PAD19  245.46,239.9 0 top
PAD20  248.28,239.9 0 top
PAD21  29.56,188.74 0 top
PAD22  32.38,188.74 0 top
PAD23  29.56,185.91 0 top
PAD24  32.38,185.91 0 top
PAD25  83.53,188.74 0 top
PAD26  86.35,188.74 0 top
PAD27  83.53,185.91 0 top
PAD28  86.35,185.91 0 top
PAD29  137.51,188.74 0 top
PAD30  140.33,188.74 0 top
PAD31  137.51,185.91 0 top
PAD32  140.33,185.91 0 top
PAD33  191.48,188.74 0 top
PAD34  194.3,188.74 0 top
PAD35  191.48,185.91 0 top
PAD36  194.3,185.91 0 top
PAD37  245.46,188.74 0 top
PAD38  248.28,188.74 0 top
PAD39  245.46,185.91 0 top
PAD40  248.28,185.91 0 top
PAD41  29.56,134.76 0 top
PAD42  32.38,134.76 0 top
PAD43  29.56,131.93 0 top
PAD44  32.38,131.94 0 top
PAD45  83.53,134.76 0 top
PAD46  86.35,134.76 0 top
PAD47  83.53,131.94 0 top
PAD48  86.35,131.94 0 top
PAD49  137.51,134.76 0 top
PAD50  140.33,134.76 0 top
PAD51  137.51,131.94 0 top
PAD52  140.33,131.94 0 top
PAD53  191.48,134.76 0 top
PAD54  194.3,134.76 0 top
PAD55  191.48,131.94 0 top
PAD56  194.3,131.94 0 top
PAD57  245.46,134.62 0 top
PAD58  248.28,134.62 0 top
PAD59  245.46,131.94 0 top
PAD60  248.28,131.94 0 top
PAD61  29.56,80.79 0 top
PAD62  32.38,80.79 0 top
PAD63  29.56,77.96 0 top
PAD64  32.38,77.96 0 top
PAD65  83.53,80.79 0 top
PAD66  86.35,80.79 0 top
PAD67  83.53,77.96 0 top
PAD68  86.35,77.96 0 top
PAD69  137.51,80.79 0 top
PAD70  140.33,80.79 0 top
PAD71  137.51,77.96 0 top
PAD72  140.33,77.96 0 top
PAD73  191.48,80.79 0 top
PAD74  194.3,80.79 0 top
PAD75  191.48,77.96 0 top
PAD76  194.3,77.96 0 top
PAD77  245.46,80.79 0 top
PAD78  248.28,80.79 0 top
PAD79  245.46,77.96 0 top
PAD80  248.28,77.96 0 top
PAD81  29.56,26.81 0 top
PAD82  32.38,26.81 0 top
PAD83  29.56,23.99 0 top
PAD84  32.38,23.99 0 top
PAD85  83.53,26.81 0 top
PAD86  86.35,26.81 0 top
PAD87  83.53,23.99 0 top
PAD88  86.35,23.99 0 top
PAD89  137.51,26.81 0 top
PAD90  140.33,26.81 0 top
PAD91  137.51,23.99 0 top
PAD92  140.33,23.99 0 top
PAD93  191.48,26.81 0 top
PAD94  194.3,26.81 0 top
PAD95  191.48,23.99 0 top
PAD96  194.3,23.99 0 top
PAD97  245.46,26.81 0 top
PAD98  248.28,26.81 0 top
PAD99  245.46,23.99 0 top
PAD100  248.28,23.99 0 top
R1  207.01,191.77 180 top
R2  96.52,132.08 180 top
R3  204.47,78.74 180 top
R4  43.18,72.39 180 top
R5  203.2,24.13 180 top
R6  207.01,186.69 0 top
R7  96.52,129.54 0 top
R8  204.47,76.2 180 bottom
R9  43.18,69.85 0 top
R10  203.2,16.51 0 top
SCL  18.7,239.89 0 top
SCL1  72.67,239.89 0 top
SCL2  126.65,239.89 0 top
SCL3  180.62,239.89 0 top
SCL4  234.6,239.89 0 top
SCL5  18.7,185.91 0 top
SCL6  72.67,185.91 0 top
SCL7  126.65,185.91 0 top
SCL8  180.62,185.91 0 top
SCL9  234.6,185.91 0 top
SCL10  18.7,131.94 0 top
SCL11  72.67,131.94 0 top
SCL12  126.65,131.94 0 top
SCL13  180.62,131.94 0 top
SCL14  234.6,131.94 0 top
SCL15  18.7,77.96 0 top
SCL16  72.67,77.96 0 top
SCL17  126.65,77.96 0 top
SCL18  180.62,77.96 0 top
SCL19  234.6,77.96 0 top
SCL20  18.7,23.99 0 top
SCL21  72.67,23.99 0 top
SCL22  126.65,23.99 0 top
SCL23  180.62,23.99 0 top
SCL24  234.6,23.99 0 top
SDA  18.7,242.71 0 top
SDA1  72.67,242.71 0 top
SDA2  126.65,242.71 0 top
SDA3  180.62,242.71 0 top
SDA4  234.6,242.71 0 top
SDA5  18.7,188.74 0 top
SDA6  72.67,188.74 0 top
SDA7  126.65,188.74 0 top
SDA8  180.62,188.74 0 top
SDA9  234.6,188.74 0 top
SDA10  18.7,134.76 0 top
SDA11  72.67,134.76 0 top
SDA12  126.65,134.76 0 top
SDA13  180.62,134.76 0 top
SDA14  234.6,134.76 0 top
SDA15  18.7,80.79 0 top
SDA16  72.67,80.79 0 top
SDA17  126.65,80.79 0 top
SDA18  180.62,80.79 0 top
SDA19  234.6,80.79 0 top
SDA20  18.7,26.81 0 top
SDA21  72.67,26.81 0 top
SDA22  126.65,26.81 0 top
SDA23  180.62,26.81 0 top
SDA24  234.6,26.81 0 top
VCC  23.99,245.45 0 top
VCC1  77.96,245.45 0 top
VCC2  131.94,245.45 0 top
VCC3  185.91,245.45 0 top
VCC4  239.89,245.45 0 top
VCC5  23.99,191.47 0 top
VCC6  77.96,191.47 0 top
VCC7  131.94,191.47 0 top
VCC8  185.91,191.47 0 top
VCC9  239.89,191.47 0 top
VCC10  23.99,137.5 0 top
VCC11  77.96,137.5 0 top
VCC12  131.94,137.5 0 top
VCC13  185.91,137.5 0 top
VCC14  239.89,137.5 0 top
VCC15  23.99,83.52 0 top
VCC16  77.96,83.52 0 top
VCC17  131.94,83.52 0 top
VCC18  185.91,83.52 0 top
VCC19  239.89,83.52 0 top
VCC20  23.99,29.55 0 top
VCC21  77.96,29.55 0 top
VCC22  131.94,29.55 0 top
VCC23  185.91,29.55 0 top
VCC24  239.89,29.55 0 top

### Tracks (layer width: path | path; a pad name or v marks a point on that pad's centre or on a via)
5V  (via drill 0.55)
  Top 0.508: IC1.18 116.84,213.36 IC1.3 111.76,201.93 v120.65,193.04 | v125.73,193.04 126.01,193.04 J8.3 | IC2.4 165.1,152.4 167.64,154.94 171.45,154.94 172.72,156.21 IC2.18 176.53,162.56 v252.73,162.56 | R2.P$1 R7.P$2 | R3.P$1 R8.P$2 | R5.P$1 R10.P$2 | R4.P$1 R9.P$2
  Bottom 0.508: J1.3 23.14,243.56 24.13,242.57 26.67,242.57 27.94,241.3 27.94,238.76 | 27.94,238.76 29.21,237.49 68.58,237.49 69.85,236.22 77.47,236.22 78.74,237.49 | 78.74,237.49 78.74,241.3 76.48,243.56 J2.3 | 78.74,237.49 80.01,236.22 130.81,236.22 132.08,237.49 132.08,242.57 131.09,243.56 J3.3 | J6.3 21.87,189.23 24.13,189.23 25.4,187.96 25.4,185.42 26.67,184.15 | 80.01,182.88 78.74,181.61 29.21,181.61 26.67,184.15 | 80.01,182.88 80.01,186.69 77.12,189.58 J7.3 | 80.01,182.88 81.28,181.61 132.08,181.61 133.35,182.88 133.35,186.69 130.46,189.58 J8.3 | J11.3 23.14,135.61 26.67,132.08 26.67,129.54 | 26.67,129.54 29.21,127 77.47,127 80.01,129.54 | 80.01,129.54 80.01,132.08 76.48,135.61 J12.3 | 80.01,129.54 82.55,127 100.33,127 | 100.33,127 130.81,127 134.62,130.81 134.62,132.08 131.09,135.61 J13.3 | J16.3 21.87,81.28 24.13,81.28 26.67,78.74 26.67,77.47 | 46.99,74.93 29.21,74.93 26.67,77.47 | 46.99,74.93 78.74,74.93 80.01,76.2 | 80.01,76.2 80.01,78.74 77.12,81.63 J17.3 | 80.01,76.2 81.28,74.93 133.35,74.93 134.62,76.2 134.62,78.74 131.73,81.63 J18.3 | J21.3 23.14,27.66 26.67,24.13 26.67,21.59 | 26.67,21.59 27.94,20.32 78.74,20.32 80.01,21.59 | 80.01,21.59 80.01,25.4 77.75,27.66 J22.3 | 80.01,21.59 81.28,20.32 132.08,20.32 133.35,21.59 | 133.35,21.59 133.35,25.4 131.09,27.66 J23.3 | 133.35,21.59 134.62,20.32 186.69,20.32 187.96,21.59 | 187.96,21.59 187.96,25.4 185.7,27.66 J24.3 | 187.96,21.59 189.23,20.32 207.01,20.32 | 207.01,20.32 240.03,20.32 241.3,21.59 | 241.3,21.59 241.3,25.4 239.04,27.66 J25.3 | 26.67,21.59 25.4,20.32 17.78,20.32 12.7,25.4 12.7,40.64 | 15.24,73.66 12.7,71.12 12.7,40.64
  Bottom 0.508: 15.24,73.66 22.86,73.66 26.67,77.47 | 15.24,73.66 12.7,76.2 12.7,101.6 | 12.7,101.6 12.7,119.38 13.97,120.65 | 26.67,129.54 17.78,120.65 13.97,120.65 | 13.97,120.65 13.97,177.8 17.78,181.61 | 17.78,181.61 25.4,181.61 26.67,182.88 26.67,184.15 | 17.78,181.61 13.97,185.42 13.97,229.87 19.05,234.95 24.13,234.95 27.94,238.76 | J19.3 186.34,81.63 189.23,78.74 189.23,76.2 191.77,73.66 208.28,73.66 | 242.57,74.93 241.3,73.66 208.28,73.66 | 242.57,74.93 242.57,78.74 239.68,81.63 J20.3 | J14.3 185.7,135.61 187.96,133.35 187.96,130.81 190.5,128.27 226.06,128.27 227.33,127 240.03,127 242.57,129.54 | 242.57,129.54 242.57,132.08 239.04,135.61 J15.3 | J9.3 186.34,189.58 187.96,187.96 187.96,184.15 189.23,182.88 198.12,182.88 199.39,184.15 210.82,184.15 | 210.82,184.15 227.33,184.15 229.87,181.61 240.03,181.61 242.57,184.15 | 242.57,184.15 242.57,187.96 240.95,189.58 J10.3 | J4.3 184.43,243.56 187.96,240.03 187.96,237.49 189.23,236.22 240.03,236.22 242.57,238.76 | 242.57,238.76 242.57,241.3 240.31,243.56 J5.3 | v120.65,193.04 v125.73,193.04 | 242.57,238.76 243.84,237.49 243.84,236.22 246.38,233.68 256.54,233.68 257.81,232.41 257.81,184.15 254,180.34 | 254,180.34 246.38,180.34 242.57,184.15 | 254,180.34 259.08,175.26 259.08,162.56 | 250.19,125.73 259.08,134.62 259.08,162.56 | 250.19,125.73 246.38,125.73 242.57,129.54 | 250.19,125.73 256.54,119.38 256.54,76.2 254,73.66 | 254,73.66 243.84,73.66 242.57,74.93 | 254,73.66 256.54,71.12 256.54,21.59 254,19.05 243.84,19.05 241.3,21.59 | v252.73,162.56 259.08,162.56 | IC3.18 106.68,50.8 102.87,50.8 100.33,48.26 IC3.5 100.33,44.45 96.52,40.64 12.7,40.64
  Bottom 0.508: ARD-5V.1 12.7,101.6 | R1.P$1 R6.P$2 210.82,184.15 | R7.P$2 100.33,127 | R4.P$1 46.99,74.93 | R10.P$2 207.01,20.32 | R8.P$2 208.28,73.66
GND  (via drill 0.55)
  other vias: 49.53,256.54 115.57,255.27 175.26,256.54 234.95,256.54 233.68,210.82 168.91,213.36 128.27,210.82 87.63,201.93 46.99,204.47 33.02,163.83 93.98,163.83 153.67,184.15 187.96,170.18 229.87,151.13 40.64,115.57 78.74,114.3 60.96,90.17 163.83,99.06 218.44,97.79 167.64,49.53 201.93,50.8 236.22,49.53 44.45,58.42 49.53,35.56
  pour Top: 0,266.7 266.7,266.7 266.7,0 0,0
  pour Bottom: 0,266.7 266.7,266.7 266.7,0 0,0
GPIO1  (via drill 0.55)
  Top 0.508: J1.1 17.78,234.74 v17.78,231.14
  Bottom 0.508: IC1.10 86.36,226.06 22.86,226.06 v17.78,231.14
GPIO2  (via drill 0.55)
  Top 0.508: v74.93,233.68 74.93,237.91 J2.1
  Bottom 0.508: IC1.11 81.28,233.68 v74.93,233.68
GPIO3  (via drill 0.55)
  Top 0.508: v123.19,233.68 124.46,234.95 128.27,234.95 129.47,236.15 J3.1
  Bottom 0.508: IC1.12 119.38,233.68 v123.19,233.68
GPIO4  (via drill 0.55)
  Top 0.508: v139.7,224.79 113.03,224.79 IC1.13
  Bottom 0.508: v139.7,224.79 146.05,224.79 157.48,236.22 181.19,236.22 J4.1
GPIO5  (via drill 0.55)
  Top 0.508: IC1.14 113.03,222.25 v139.7,222.25 | v231.14,233.68 233.68,236.22 236.22,236.22 237.42,237.42 J5.1
  Bottom 0.508: v231.14,233.68 158.75,233.68 147.32,222.25 v139.7,222.25
GPIO6
  Top 0.508: IC1.15 106.68,213.36 36.83,213.36 13.97,190.5 13.97,185.42 16.51,182.88 19.9,182.88 J6.1
GPIO7  (via drill 0.55)
  Top 0.508: IC1.16 111.76,214.63 107.95,210.82 74.93,210.82 v52.07,187.96
  Bottom 0.508: v52.07,187.96 57.15,182.88 73.87,182.88 J7.1
GPIO8  (via drill 0.55)
  Top 0.508: v115.57,194.31 v115.57,187.96
  Bottom 0.508: IC1.17 114.3,213.36 115.57,212.09 118.11,212.09 120.65,209.55 120.65,199.39 v115.57,194.31 | v115.57,187.96 120.65,182.88 127.85,182.88 J8.1
GPIO9
  Bottom 0.254: IC2.10 172.72,179.07 180.34,179.07 183.44,182.17 J9.1
GPIO10  (via drill 0.55)
  Top 0.254: v223.52,181.61 224.79,182.88 235.8,182.88 J10.1
  Bottom 0.254: IC2.11 173.99,177.8 219.71,177.8 v223.52,181.61
GPIO11  (via drill 0.55)
  Top 0.254: IC2.12 157.48,157.48 156.21,156.21 134.62,156.21 v132.08,153.67
  Bottom 0.254: v132.08,153.67 123.19,144.78 22.86,144.78 16.51,138.43 16.51,130.81 17.78,129.54 20.53,129.54 J11.1
GPIO12  (via drill 0.55)
  Top 0.254: IC2.13 160.02,156.21 158.75,154.94 135.89,154.94 v132.08,151.13 | v52.07,133.35 v52.07,138.43
  Bottom 0.254: v132.08,151.13 124.46,143.51 57.15,143.51 v52.07,138.43 | v52.07,133.35 55.88,129.54 74.51,129.54 J12.1
GPIO13  (via drill 0.55)
  Top 0.254: IC2.14 162.56,156.21 160.02,153.67 137.16,153.67 v132.08,148.59 | v121.92,138.43 119.38,135.89 v119.38,133.35
  Bottom 0.254: v132.08,148.59 v121.92,138.43 | v119.38,133.35 123.19,129.54 128.48,129.54 J13.1
GPIO14  (via drill 0.55)
  Top 0.254: v168.91,137.16 171.45,134.62 v171.45,133.35
  Bottom 0.254: IC2.15 165.1,156.21 163.83,154.94 151.13,154.94 149.86,153.67 149.86,149.86 162.56,137.16 v168.91,137.16 | v171.45,133.35 175.26,129.54 182.46,129.54 J14.1
GPIO15  (via drill 0.55)
  Top 0.254: v222.25,139.7 226.06,135.89 v226.06,133.35
  Bottom 0.254: IC2.16 167.64,156.21 168.91,154.94 207.01,154.94 v222.25,139.7 | v226.06,133.35 229.87,129.54 236.43,129.54 J15.1
GPIO16  (via drill 0.55)
  Top 0.508: IC2.17 170.18,161.29 137.16,161.29 v132.08,156.21 | v17.78,147.32 10.16,139.7 v10.16,132.08 | v10.16,76.2 11.43,74.93 19.9,74.93 J16.1
  Bottom 0.508: v132.08,156.21 123.19,147.32 v17.78,147.32 | v10.16,132.08 v10.16,76.2
GPIO17  (via drill 0.55)
  Top 0.508: v72.39,69.85 72.39,73.45 J17.1
  Bottom 0.508: IC3.10 87.63,54.61 v72.39,69.85
GPIO18  (via drill 0.55)
  Top 0.508: v121.92,71.12 124.46,71.12 129.47,76.13 J18.1
  Bottom 0.508: IC3.11 92.71,60.96 102.87,71.12 v121.92,71.12
GPIO19  (via drill 0.55)
  Top 0.508: IC3.12 95.25,58.42 97.79,60.96 v139.7,60.96
  Bottom 0.508: J19.1 180.55,73.66 161.29,73.66 148.59,60.96 v139.7,60.96
GPIO20  (via drill 0.55)
  Top 0.508: IC3.13 97.79,57.15 99.06,58.42 v139.7,58.42 | v213.36,69.85 217.17,73.66 234.53,73.66 J20.1
  Bottom 0.508: v213.36,69.85 162.56,69.85 151.13,58.42 v139.7,58.42
GPIO21
  Top 0.254: IC3.14 100.33,53.34 99.06,52.07 34.29,52.07 12.7,30.48 12.7,25.4 16.51,21.59 20.53,21.59 J21.1
GPIO22  (via drill 0.55)
  Top 0.254: IC3.15 102.87,52.07 101.6,50.8 83.82,50.8 67.31,34.29 v67.31,25.4
  Bottom 0.254: v67.31,25.4 68.58,24.13 68.58,22.86 69.85,21.59 74.51,21.59 J22.1
GPIO23  (via drill 0.55)
  Top 0.254: IC3.16 105.41,52.07 107.95,49.53 v115.57,49.53 | v120.65,39.37 120.65,29.21 v118.11,26.67
  Bottom 0.254: v115.57,49.53 120.65,44.45 v120.65,39.37 | v118.11,26.67 118.11,22.86 119.38,21.59 128.48,21.59 J23.1
GPIO24  (via drill 0.55)
  Top 0.254: IC3.17 107.95,53.34 109.22,52.07 129.54,52.07 v139.7,41.91 | v171.45,30.48 173.99,27.94 v173.99,25.4
  Bottom 0.254: v139.7,41.91 151.13,30.48 v171.45,30.48 | v173.99,25.4 177.8,21.59 182.46,21.59 J24.1
GPIO25  (via drill 0.55)
  Top 0.254: ARD-DIG-PIN.1 124.46,96.52 v139.7,111.76 | v251.46,101.6 256.54,96.52 256.54,21.59 247.65,12.7 v241.3,12.7 | v236.22,17.78 236.22,21.38 J25.1
  Bottom 0.254: v139.7,111.76 241.3,111.76 v251.46,101.6 | v241.3,12.7 v236.22,17.78
N$6  (via drill 0.55)
  other vias: 46.99,219.71
N$11  (via drill 0.55)
  other vias: 222.25,190.5
SCL
  Top 0.254: SCL.1 16.51,242.08 16.51,243.84 20.32,247.65 27.44,247.65 PAD2.1 51.93,242.71 54.75,239.89 71.26,239.89 | 71.26,239.89 69.85,241.3 69.85,243.84 73.66,247.65 81.42,247.65 PAD6.1 86.5,242.57 102.87,242.57 105.55,239.89 SCL2.1 124.6,239.89 123.19,241.3 123.19,243.84 127,247.65 138.43,247.65 140.33,245.75 PAD10.1 140.47,242.57 143.51,242.57 | 71.26,239.89 SCL1.1 | 179.21,239.89 177.8,241.3 177.8,243.84 181.61,247.65 190.5,247.65 194.3,243.85 PAD14.1 194.44,242.57 213.36,242.57 216.04,239.89 SCL4.1 232.55,239.89 231.14,241.3 231.14,243.84 234.95,247.65 243.84,247.65 248.28,243.21 PAD18.1 | 179.21,239.89 SCL3.1 | SCL5.1 16.02,185.91 15.24,186.69 15.24,189.23 20.32,194.31 27.94,194.31 32.38,189.87 PAD22.1 33.16,187.96 44.45,187.96 46.5,185.91 69.36,185.91 | 69.36,185.91 68.58,186.69 68.58,189.23 73.66,194.31 82.55,194.31 86.35,190.51 PAD26.1 104.63,188.74 107.46,185.91 SCL7.1 123.97,185.91 123.19,186.69 123.19,194.31 | 69.36,185.91 SCL6.1 | 135.89,194.31 140.33,189.87 PAD30.1 141.1,187.96 146.05,187.96 | 123.19,194.31 135.89,194.31 | 177.31,185.91 176.53,186.69 176.53,189.23 181.61,194.31 189.23,194.31 194.3,189.24 PAD34.1 | 177.31,185.91 SCL8.1 | PAD38.1 248.28,189.87 243.84,194.31 236.22,194.31 231.14,189.23 231.14,186.69 231.92,185.91 SCL9.1 216.68,185.91 213.85,188.74 PAD34.1 | SCL10.1 15.38,131.94 15.24,132.08 15.24,134.62 20.32,139.7 27.94,139.7 32.38,135.26 PAD42.1 44.31,134.76 48.4,130.67 68.72,130.67 | 68.72,130.67 68.58,130.81 68.58,135.89 73.66,140.97 81.28,140.97 86.35,135.9 PAD46.1 | 68.72,130.67 71.4,130.67 SCL11.1
  Top 0.254: 128.27,140.97 135.89,140.97 140.33,136.53 PAD50.1 147.32,134.76 | 128.27,140.97 123.19,135.89 123.19,132.08 124.6,130.67 | 124.6,130.67 125.38,130.67 SCL12.1 | 181.61,140.97 189.23,140.97 194.3,135.9 PAD54.1 213.22,134.76 217.31,130.67 232.55,130.67 | 181.61,140.97 177.8,137.16 177.8,132.08 179.21,130.67 | 179.21,130.67 179.35,130.67 SCL13.1 | PAD58.1 248.28,136.53 243.84,140.97 236.22,140.97 231.14,135.89 231.14,132.08 232.55,130.67 | 232.55,130.67 233.33,130.67 SCL14.1 | PAD62.1 32.38,81.92 27.94,86.36 20.32,86.36 15.24,81.28 15.24,78.74 16.02,77.96 SCL15.1 | 134.62,90.17 140.33,84.46 PAD70.1 143.51,80.79 | 134.62,90.17 129.54,90.17 123.19,83.82 123.19,78.74 123.97,77.96 SCL17.1 107.46,77.96 104.63,80.79 PAD66.1 86.35,81.29 81.28,86.36 73.66,86.36 69.85,82.55 69.85,78.74 70.63,77.96 SCL16.1 51.58,77.96 48.75,80.79 PAD62.1 | 178.58,77.96 177.8,78.74 177.8,81.28 182.88,86.36 190.5,86.36 194.3,82.56 PAD74.1 | 178.58,77.96 SCL18.1 | PAD78.1 248.28,81.92 243.84,86.36 236.22,86.36 231.14,81.28 231.14,78.74 231.92,77.96 SCL19.1 216.68,77.96 213.85,80.79 PAD74.1 | SCL20.1 16.65,23.99 15.24,25.4 15.24,27.94 19.05,31.75 27.94,31.75 32.38,27.31 PAD82.1 50.66,26.81 54.75,22.72 69.99,22.72 | 69.99,22.72 69.85,22.86 69.85,27.94 73.66,31.75 82.55,31.75 86.35,27.95 PAD86.1 86.5,26.67 104.14,26.67 106.82,23.99 SCL22.1 124.6,23.99 123.19,25.4 123.19,27.94 | SCL21.1 71.4,22.72 69.99,22.72 | 135.89,31.75 140.33,27.31 PAD90.1 140.47,26.67 161.29,26.67 163.97,23.99 179.21,23.99 | 123.19,27.94 127,31.75 135.89,31.75 | 179.21,23.99 177.8,25.4 177.8,27.94 181.61,31.75 190.5,31.75 194.3,27.95 PAD94.1 194.44,26.67
  Top 0.254: 179.21,23.99 SCL23.1 | PAD98.1 248.28,28.58 245.11,31.75 234.95,31.75 231.14,27.94 231.14,25.4 232.55,23.99 SCL24.1 216.04,23.99 213.36,26.67 194.44,26.67 | 143.51,242.57 158.75,242.57 161.43,239.89 179.21,239.89 | 146.05,187.96 157.48,187.96 159.53,185.91 177.31,185.91 | PAD46.1 104,134.76 108.09,130.67 124.6,130.67 | 147.32,134.76 159.88,134.76 163.97,130.67 179.21,130.67 | 143.51,80.79 159.24,80.79 162.07,77.96 178.58,77.96 | 143.51,80.79 143.51,39.37 135.89,31.75 | 134.62,90.17 134.62,99.06 147.32,111.76 147.32,121.92 | 147.32,121.92 147.32,134.76 | 128.27,140.97 128.27,158.75 146.05,176.53 146.05,187.96 | 135.89,194.31 137.16,195.58 137.16,208.28 143.51,214.63 143.51,242.57 | IC1.1 119.38,205.74 119.38,198.12 123.19,194.31 | IC2.1 181.61,142.24 181.61,140.97 | IC3.1 118.11,46.99 123.19,41.91 123.19,27.94 | ARD-SCL.1 147.32,121.92 | R2.P$2 89.04,132.08 PAD46.1 | R1.P$2 197.34,191.77 PAD34.1 | R3.P$2 196.36,78.74 PAD74.1 | R5.P$2 196.99,24.13 194.44,26.67 | R4.P$2 35.56,76.2 35.56,78.74 33.51,80.79 PAD62.1
SDA
  Top 0.254: R7.P$1 88.75,129.54 PAD48.1 | R6.P$1 195.08,186.69 PAD36.1 | R8.P$1 196.07,76.2 PAD76.1 | R10.P$1 194.3,21.6 PAD96.1 | R9.P$1 32.38,76.84 PAD64.1
  Bottom 0.254: PAD4.1 34.29,241.8 34.29,243.84 | 34.29,243.84 34.29,245.11 31.75,247.65 22.86,247.65 18.7,243.49 SDA.1 | PAD8.1 88.9,242.44 88.9,243.84 | 88.9,243.84 88.9,245.11 86.36,247.65 76.2,247.65 72.67,244.12 SDA1.1 72.53,242.57 53.34,242.57 52.07,243.84 34.29,243.84 | 143.51,243.84 143.51,243.07 PAD12.1 140.33,231.77 134.62,226.06 134.62,194.31 | 143.51,243.84 143.51,245.11 140.97,247.65 129.54,247.65 126.65,244.76 SDA2.1 126.51,242.57 105.41,242.57 104.14,243.84 88.9,243.84 | PAD16.1 198.12,243.71 198.12,245.11 | 198.12,245.11 198.12,246.38 196.85,247.65 184.15,247.65 180.62,244.12 SDA3.1 180.48,242.57 160.02,242.57 158.75,243.84 143.51,243.84 | PAD20.1 251.46,243.08 251.46,246.38 250.19,247.65 238.76,247.65 234.6,243.49 SDA4.1 234.46,242.57 215.9,242.57 213.36,245.11 198.12,245.11 | PAD24.1 35.56,189.09 35.56,190.5 | SDA5.1 18.7,190.15 22.86,194.31 34.29,194.31 35.56,193.04 35.56,190.5 | PAD28.1 86.85,185.91 90.17,189.23 90.17,190.5 | 90.17,190.5 90.17,191.77 87.63,194.31 76.2,194.31 72.67,190.78 SDA6.1 61.45,188.74 59.69,190.5 35.56,190.5 | 143.51,190.5 143.51,189.09 PAD32.1 140.33,169.54 134.62,163.83 134.62,140.97 | 143.51,190.5 143.51,191.77 140.97,194.31 134.62,194.31 | 134.62,194.31 130.81,194.31 126.65,190.15 SDA7.1 122.41,188.74 120.65,190.5 106.68,190.5 | PAD40.1 249.41,185.91 252.73,189.23 252.73,191.77 250.19,194.31 233.68,194.31 233.33,193.96 | 233.33,193.96 233.33,190.5 234.6,189.23 SDA9.1 | 233.33,193.96 233.33,194.31 202.7,194.31 PAD36.1 198.12,189.73 198.12,190.5 194.31,194.31 184.15,194.31 180.62,190.78 SDA8.1 159.24,188.74 157.48,190.5 143.51,190.5
  Bottom 0.254: PAD44.1 35.56,135.12 35.56,135.89 | SDA10.1 18.7,135.54 22.86,139.7 33.02,139.7 35.56,137.16 35.56,135.89 | PAD48.1 90.17,135.75 90.17,135.89 | 90.17,135.89 90.17,138.43 87.63,140.97 76.2,140.97 72.67,137.44 SDA11.1 72.53,134.62 55.88,134.62 54.61,135.89 35.56,135.89 | 134.62,140.97 140.97,140.97 143.51,138.43 143.51,135.89 | 134.62,140.97 130.81,140.97 126.65,136.81 SDA12.1 126.51,134.62 109.22,134.62 107.95,135.89 90.17,135.89 | 143.51,135.89 143.51,135.12 PAD52.1 140.33,120.01 134.62,114.3 | PAD56.1 198.12,135.75 198.12,135.89 | 198.12,135.89 198.12,138.43 195.58,140.97 184.15,140.97 180.62,137.44 SDA13.1 179.49,135.89 175.26,135.89 | PAD60.1 252.73,136.39 252.73,138.43 250.19,140.97 237.49,140.97 234.6,138.08 SDA14.1 233.47,135.89 198.12,135.89 | PAD64.1 35.56,81.14 35.56,81.28 | SDA15.1 18.7,82.2 22.86,86.36 33.02,86.36 35.56,83.82 35.56,81.28 | PAD68.1 90.17,81.78 90.17,82.55 | 72.67,81.28 72.67,82.83 76.2,86.36 88.9,86.36 90.17,85.09 90.17,82.55 | 72.67,81.28 SDA16.1 | 143.51,81.28 143.51,81.14 PAD72.1 140.33,69.21 135.89,64.77 135.89,31.75 | 143.51,81.28 143.51,82.55 135.89,90.17 134.62,90.17 | 134.62,90.17 126.65,82.2 126.65,81.28 | 126.65,81.28 SDA17.1 | PAD76.1 198.12,81.78 198.12,82.55 | 180.62,81.28 180.62,81.56 185.42,86.36 195.58,86.36 198.12,83.82 198.12,82.55 | 180.62,81.28 SDA18.1 | PAD80.1 251.46,81.14 251.46,83.82 248.92,86.36 238.76,86.36 234.6,82.2 SDA19.1 218.93,80.79 217.17,82.55 198.12,82.55 | PAD84.1 35.56,27.17 35.56,27.94 | SDA20.1 18.7,28.86 21.59,31.75 33.02,31.75 35.56,29.21 35.56,27.94 | PAD88.1 88.9,26.54 88.9,29.21 | 88.9,29.21 88.9,30.48 87.63,31.75 76.2,31.75 72.67,28.22 SDA21.1 71.54,27.94 35.56,27.94
  Bottom 0.254: PAD92.1 143.51,27.17 143.51,27.94 | 135.89,31.75 142.24,31.75 143.51,30.48 143.51,27.94 | 135.89,31.75 129.54,31.75 126.65,28.86 SDA22.1 126.51,26.67 121.92,26.67 119.38,29.21 | PAD96.1 196.85,26.54 196.85,27.94 | 196.85,27.94 196.85,29.21 194.31,31.75 184.15,31.75 180.62,28.22 SDA23.1 180.48,26.67 176.53,26.67 175.26,27.94 143.51,27.94 | PAD100.1 250.19,25.9 250.19,29.21 247.65,31.75 237.49,31.75 234.6,28.86 SDA24.1 234.46,26.67 215.9,26.67 214.63,27.94 196.85,27.94 | 88.9,29.21 119.38,29.21 | 35.56,81.28 72.67,81.28 | 90.17,82.55 107.95,82.55 109.22,81.28 126.65,81.28 | 143.51,81.28 180.62,81.28 | 175.26,135.89 143.51,135.89 | 90.17,190.5 106.68,190.5 | 134.62,114.3 134.62,90.17 | IC1.2 114.3,205.74 106.68,198.12 106.68,190.5 | IC2.2 175.26,146.05 175.26,135.89 | IC3.2 119.38,35.56 119.38,29.21 | ARD-SDA.1 132.08,116.84 134.62,114.3
VCC  (via drill 0.55)
  Top 0.508: PAD1.1 25.4,242.71 | 78.74,242.71 PAD5.1 | 134.62,242.57 137.37,242.57 PAD9.1 | 187.96,242.57 191.34,242.57 PAD13.1 | 241.3,242.57 245.32,242.57 PAD17.1 | PAD21.1 26.67,188.74 | 26.67,188.74 25.89,188.74 23.99,190.64 VCC5.1 | 80.5,188.74 PAD25.1 | 133.84,188.74 PAD29.1 | 188.45,188.74 PAD33.1 | 241.79,188.74 PAD37.1 | 26.67,134.62 29.42,134.62 PAD41.1 | 80.01,134.62 83.39,134.62 PAD45.1 | 134.62,134.62 137.37,134.62 PAD49.1 | 187.96,134.62 191.34,134.62 PAD53.1 | 242.57,134.62 PAD57.1 | 25.89,80.79 PAD61.1 | 80.01,80.79 79.23,80.79 77.96,82.06 VCC16.1 | 80.01,80.79 PAD65.1 | 133.84,80.79 PAD69.1 | 188.45,80.79 PAD73.1 | 241.79,80.79 PAD77.1 | 26.67,26.67 25.4,26.67 23.99,28.08 VCC20.1 | 26.67,26.67 29.42,26.67 PAD81.1 | 80.01,26.67 83.39,26.67 PAD85.1 | 133.35,26.67 137.37,26.67 PAD89.1 | 187.96,26.67 191.34,26.67 PAD93.1 | 241.3,26.67 245.32,26.67 PAD97.1 | 25.4,236.22 25.4,242.71 | 25.4,236.22 7.62,218.44 7.62,177.8 | 26.67,20.32 24.13,17.78 17.78,17.78 7.62,27.94 7.62,72.39 | 26.67,26.67 26.67,20.32 | 7.62,177.8 7.62,127 | 7.62,127 7.62,72.39 | 25.89,80.79 25.89,75.42 | 25.89,75.42 22.86,72.39 7.62,72.39 | 26.67,134.62 26.67,129.54 | 7.62,127 24.13,127 26.67,129.54 | 26.67,188.74 26.67,180.34 | 26.67,180.34 24.13,177.8 7.62,177.8 | 26.67,20.32 29.21,17.78 76.2,17.78 80.01,21.59 | 80.01,26.67 80.01,21.59 | 80.01,21.59 83.82,17.78 132.08,17.78 133.35,19.05 | 133.35,19.05 133.35,26.67 | 133.35,19.05 134.62,17.78 185.42,17.78 187.96,20.32 | 187.96,26.67 187.96,20.32 | 187.96,20.32 194.31,13.97 236.22,13.97 241.3,19.05 241.3,26.67 | 25.89,75.42 34.01,67.31 72.39,67.31 80.01,74.93 | 80.01,74.93 80.01,80.79 | 80.01,74.93 87.63,67.31 135.89,67.31
  Top 0.508: 133.84,80.79 133.84,75.42 130.81,72.39 135.89,67.31 | 135.89,67.31 v139.7,63.5 | v147.32,63.5 156.21,72.39 185.42,72.39 188.45,75.42 | 188.45,80.79 188.45,75.42 | 188.45,75.42 196.57,67.31 232.41,67.31 241.79,76.69 241.79,80.79 | 25.4,236.22 31.75,229.87 76.2,229.87 81.28,234.95 | 78.74,242.71 78.74,237.49 81.28,234.95 | 81.28,234.95 85.09,231.14 130.81,231.14 133.35,233.68 | 134.62,242.57 134.62,238.76 132.72,236.85 134.62,234.95 133.35,233.68 | 187.96,237.49 180.34,229.87 v147.32,229.87 | 187.96,242.57 187.96,237.49 | v139.7,227.33 133.35,233.68 | 187.96,237.49 194.31,231.14 234.95,231.14 241.3,237.49 241.3,242.57 | 26.67,180.34 29.21,177.8 49.53,177.8 52.07,180.34 77.47,180.34 80.5,183.37 | 80.5,188.74 80.5,183.37 | 80.5,183.37 83.54,180.34 130.81,180.34 133.84,183.37 | 133.84,183.37 133.84,188.74 | 133.84,183.37 134.13,183.37 137.16,180.34 v143.51,180.34 | v149.86,180.34 185.42,180.34 188.45,183.37 | 188.45,188.74 188.45,183.37 | 188.45,183.37 191.49,180.34 238.76,180.34 241.79,183.37 241.79,188.74 | 26.67,129.54 29.21,127 77.47,127 80.01,129.54 | 80.01,134.62 80.01,129.54 | 80.01,129.54 82.55,127 130.81,127 134.62,130.81 | 134.62,134.62 134.62,130.81 | 134.62,130.81 138.43,127 v143.51,127 | v151.13,127 185.42,127 187.96,129.54 | 187.96,129.54 187.96,134.62 | 187.96,129.54 190.5,127 240.03,127 242.57,129.54 242.57,134.62 | 25.4,242.71 25.4,244.03 VCC.1 | 78.74,242.71 78.74,244.67 VCC1.1 | VCC2.1 131.94,245.25 134.62,242.57 | VCC3.1 185.91,244.62 187.96,242.57 | VCC4.1 239.89,243.98 241.3,242.57 | 80.5,188.74 77.96,191.28 VCC6.1 | 133.84,188.74 131.94,190.64 VCC7.1 | 188.45,188.74 185.91,191.28 VCC8.1
  Top 0.508: 241.79,188.74 239.89,190.64 VCC9.1 | VCC14.1 239.89,137.3 242.57,134.62 | VCC13.1 185.91,136.67 187.96,134.62 | VCC12.1 131.94,137.3 134.62,134.62 | VCC11.1 77.96,136.67 80.01,134.62 | VCC10.1 23.99,137.3 26.67,134.62 | 25.89,80.79 23.99,82.69 VCC15.1 | 133.84,80.79 131.94,82.69 VCC17.1 131.94,85.23 v129.54,87.63 | 188.45,80.79 185.91,83.33 VCC18.1 | 241.79,80.79 239.89,82.69 VCC19.1 | VCC21.1 77.96,28.72 80.01,26.67 | VCC22.1 131.94,28.08 133.35,26.67 | VCC23.1 185.91,28.72 187.96,26.67 | VCC24.1 239.89,28.08 241.3,26.67
  Bottom 0.508: v139.7,63.5 v147.32,63.5 | v139.7,227.33 144.78,227.33 v147.32,229.87 | v143.51,180.34 v149.86,180.34 | v143.51,127 v151.13,127 | ARD-VCC.1 129.54,99.06 v129.54,87.63

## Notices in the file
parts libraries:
SparkFun-Connectors: Licensing: Creative Commons ShareAlike 4.0 International - https://creativecommons.org/licenses/by-sa/4.0
